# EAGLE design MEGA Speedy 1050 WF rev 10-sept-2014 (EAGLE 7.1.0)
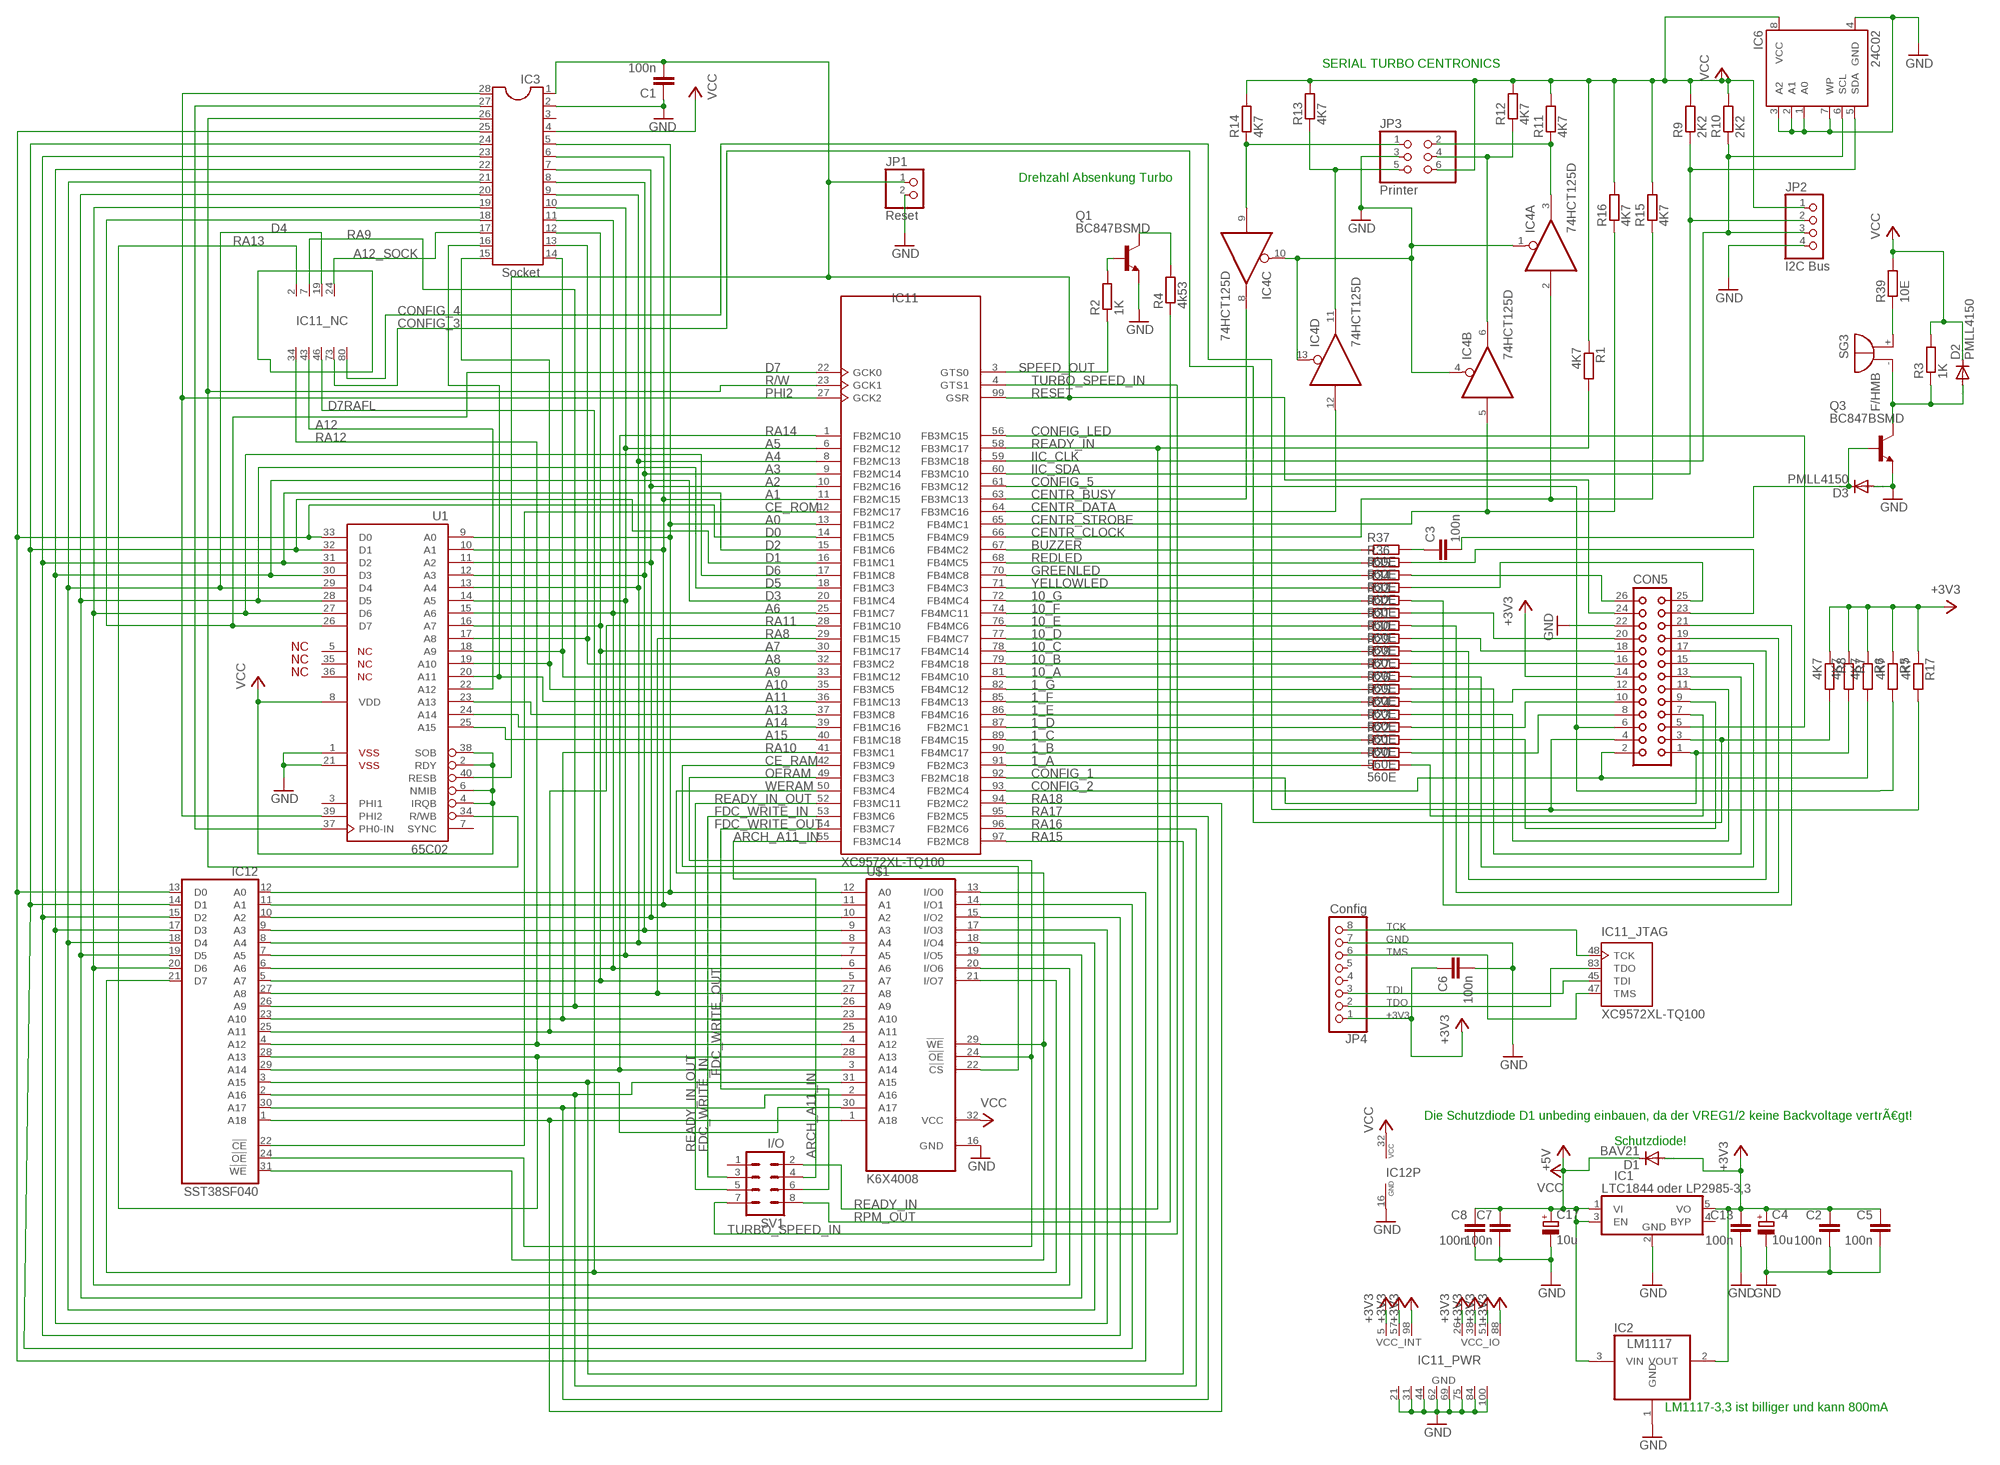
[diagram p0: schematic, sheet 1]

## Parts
C1  100n  C-EUC0805  [C0805]
C2  100n  C-EUC0805  [C0805]
C3  100n  C-EUC0805  [C0805]
C4  10u  CPOL-EUD/7343-31W  [D/7343-31W]
C5  100n  C-EUC0805  [C0805]
C6  100n  C-EUC0805  [C0805]
C7  100n  C-EUC0805  [C0805]
C8  100n  C-EUC0805  [C0805]
C13  100n  C-EUC0805  [C0805]
C17  10u  CPOL-EUD/7343-31W  [D/7343-31W]
CON5  CON26L  [CON26L]
D1  BAV21  PMLL4150  [SOD80C]
D2  PMLL4150  [SOD80C]
D3  PMLL4150  [SOD80C]
IC1  LTC1844 oder LP2985-3,3  LTC1844  [SOT23/5]
IC2  LM1117  REG1117  [SOT223]
IC3  Socket  DIL28  [DIL28-6]
IC4  74HCT125D  [SO14]
IC6  24C02  AT24C  [SOIC8]
IC11  XC9572XL-TQ100  [TQ100]
IC12  SST38SF040  AM29F040J  [PLCC32R]
JP1  Reset  PINHD-1X2  [1X02]
JP2  I2C Bus  PINHD-1X4  [1X04]
JP3  Printer  PINHD-2X3  [2X03]
JP4  Config  PINHD-1X8  [1X08]
Q1  BC847BSMD  [SOT23]
Q3  BC847BSMD  [SOT23]
R1  4K7  R-EU_M0805  [M0805]
R2  1K  R-EU_M0805  [M0805]
R3  1K  R-EU_M0805  [M0805]
R4  4k53  R-EU_M0805  [M0805]
R5  4K7  R-EU_M0805  [M0805]
R6  4K7  R-EU_M0805  [M0805]
R7  4K7  R-EU_M0805  [M0805]
R8  4K7  R-EU_M0805  [M0805]
R9  2K2  R-EU_M0805  [M0805]
R10  2K2  R-EU_M0805  [M0805]
R11  4K7  R-EU_M0805  [M0805]
R12  4K7  R-EU_M0805  [M0805]
R13  4K7  R-EU_M0805  [M0805]
R14  4K7  R-EU_M0805  [M0805]
R15  4K7  R-EU_M0805  [M0805]
R16  4K7  R-EU_M0805  [M0805]
R17  4K7  R-EU_M0805  [M0805]
R20  560E  R-EU_M0805  [M0805]
R21  560E  R-EU_M0805  [M0805]
R22  560E  R-EU_M0805  [M0805]
R23  560E  R-EU_M0805  [M0805]
R24  560E  R-EU_M0805  [M0805]
R25  560E  R-EU_M0805  [M0805]
R26  560E  R-EU_M0805  [M0805]
R27  560E  R-EU_M0805  [M0805]
R28  560E  R-EU_M0805  [M0805]
R29  560E  R-EU_M0805  [M0805]
R30  560E  R-EU_M0805  [M0805]
R31  560E  R-EU_M0805  [M0805]
R32  560E  R-EU_M0805  [M0805]
R33  560E  R-EU_M0805  [M0805]
R34  560E  R-EU_M0805  [M0805]
R35  560E  R-EU_M0805  [M0805]
R36  560E  R-EU_M0805  [M0805]
R37  560E  R-EU_M0805  [M0805]
R39  10E  R-EU_M0805  [M0805]
SG3  F/HMB  [F/HMB]
SV1  I/O  MA04-2  [MA04-2]
U1  65C02  G65SC02P  [DIP-40]
U$1  K6X4008  [SOP32L]

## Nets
1_A: IC11.91(FB2MC3) R20.1
1_B: IC11.90(FB4MC17) R21.1
1_C: IC11.89(FB4MC15) R22.1
1_D: IC11.87(FB2MC1) R23.1
1_E: IC11.86(FB4MC16) R24.1
1_F: IC11.85(FB4MC13) R25.1
1_G: IC11.82(FB4MC12) R26.1
10_A: IC11.81(FB4MC10) R27.1
10_B: IC11.79(FB4MC18) R28.1
10_C: IC11.78(FB4MC14) R29.1
10_D: IC11.77(FB4MC7) R30.1
10_E: IC11.76(FB4MC6) R31.1
10_F: IC11.74(FB4MC11) R32.1
10_G: IC11.72(FB4MC4) R33.1
+3V3: C2.1 C4.+ C5.1 C6.1 C13.1 CON5.14 D1.A IC1.5(VO) IC2.2(VOUT) IC11.5(VCC_INT) IC11.26(VCC_IO) IC11.38(VCC_IO) IC11.51(VCC_IO) IC11.57(VCC_INT) IC11.88(VCC_IO) IC11.98(VCC_INT) JP4.1 R5.1 R6.1 R7.1 R8.1 R17.1
A0: IC3.5 IC11.13(FB1MC2) IC12.12(A0) U1.9(A0) U$1.12(A0)
A1: IC3.6 IC11.11(FB2MC15) IC12.11(A1) U1.10(A1) U$1.11(A1)
A2: IC3.7 IC11.10(FB2MC16) IC12.10(A2) U1.11(A2) U$1.10(A2)
A3: IC3.8 IC11.9(FB2MC14) IC12.9(A3) U1.12(A3) U$1.9(A3)
A4: IC3.9 IC11.8(FB2MC13) IC12.8(A4) U1.13(A4) U$1.8(A4)
A5: IC3.10 IC11.6(FB2MC12) IC12.7(A5) U1.14(A5) U$1.7(A5)
A6: IC3.11 IC11.25(FB1MC7) IC12.6(A6) U1.15(A6) U$1.6(A6)
A7: IC3.12 IC11.30(FB1MC17) IC12.5(A7) U1.16(A7) U$1.5(A7)
A8: IC3.13 IC11.32(FB3MC2) U1.17(A8)
A9: IC3.14 IC11.33(FB1MC12) U1.18(A9)
A10: IC3.15 IC11.35(FB3MC5) U1.19(A10)
A11: IC3.16 IC11.36(FB1MC13) U1.20(A11)
A12: IC11.43(NC) U1.22(A12)
A12_SOCK: IC3.17 IC11.24(NC)
A13: IC11.37(FB3MC8) U1.23(A13)
A14: IC11.39(FB1MC16) U1.24(A14)
A15: IC11.40(FB1MC18) U1.25(A15)
ARCH_A11_IN: IC11.55(FB3MC14) SV1.4
BUZZER: IC11.67(FB4MC2) R37.1
CE_RAM: IC11.42(FB3MC9) U$1.22(!CS)
CE_ROM: IC11.12(FB2MC17) IC12.22(!CE)
CENTR_BUSY: IC4.8(C:O) IC11.63(FB3MC13)
CENTR_CLOCK: IC4.2(A:I) IC11.66(FB4MC9) R15.1
CENTR_DATA: IC4.12(D:I) IC11.64(FB3MC16)
CENTR_STROBE: IC4.5(B:I) IC11.65(FB4MC1) R16.1
CONFIG_1: CON5.1 IC11.92(FB2MC18) R7.2
CONFIG_2: CON5.2 IC11.93(FB2MC4) R6.2
CONFIG_3: CON5.3 IC11.73(NC) R8.2
CONFIG_4: CON5.4 IC11.80(NC) R17.2
CONFIG_5: CON5.6 IC11.61(FB3MC12) R5.2
CONFIG_LED: CON5.5 IC11.56(FB3MC15)
D0: IC3.25 IC11.14(FB1MC5) IC12.13(D0) U1.33(D0) U$1.13(I/O0)
D1: IC3.24 IC11.16(FB1MC1) IC12.14(D1) U1.32(D1) U$1.14(I/O1)
D2: IC3.23 IC11.15(FB1MC6) IC12.15(D2) U1.31(D2) U$1.15(I/O2)
D3: IC3.22 IC11.20(FB1MC4) IC12.17(D3) U1.30(D3) U$1.17(I/O3)
D4: IC3.21 IC11.19(NC) IC12.18(D4) U1.29(D4) U$1.18(I/O4)
D5: IC3.20 IC11.18(FB1MC3) IC12.19(D5) U1.28(D5) U$1.19(I/O5)
D6: IC3.19 IC11.17(FB1MC8) IC12.20(D6) U1.27(D6) U$1.20(I/O6)
D7: IC3.18 IC11.22(GCK0) U1.26(D7)
D7RAFL: IC11.46(NC) IC12.21(D7) U$1.21(I/O7)
FDC_WRITE_IN: IC11.53(FB3MC6) SV1.3
FDC_WRITE_OUT: IC11.54(FB3MC7) SV1.6
GND: C1.1 C2.2 C4.- C5.2 C6.2 C7.2 C8.2 C13.2 C17.- CON5.22 D3.A IC1.2(GND) IC2.1(GND) IC3.2 IC4.1(A:OE) IC4.4(B:OE) IC4.10(C:OE) IC4.13(D:OE) IC6.1(A0) IC6.2(A1) IC6.3(A2) IC6.4(GND) IC6.7(WP) IC11.21(GND) IC11.31(GND) IC11.44(GND) IC11.62(GND) IC11.69(GND) IC11.75(GND) IC11.84(GND) IC11.100(GND) IC12.16(GND) JP1.2 JP2.4 JP3.3 JP4.7 Q1.2(E) Q3.2(E) U1.1(VSS$1) U1.21(VSS$2) U$1.16(GND)
GREENLED: IC11.70(FB4MC8) R35.1
IIC_CLK: IC6.6(SCL) IC11.59(FB3MC18) JP2.3 R10.1
IIC_SDA: IC6.5(SDA) IC11.60(FB3MC10) JP2.2 R9.1
N$2: Q1.1(B) R2.2
N$7: Q1.3(C) R4.2
N$8: R39.1 SG3.+
N$11: D2.A Q3.3(C) R3.1 SG3.-
N$36: IC3.27 U1.37(PH0-IN)
N$41: IC4.6(B:O) JP3.4 R12.1
N$42: IC4.3(A:O) JP3.2 R11.1
N$43: IC4.9(C:I) JP3.1 R14.1
N$44: IC4.11(D:O) JP3.5 R13.1
N$86: C3.1 R37.2
N$96: C3.2 D3.C Q3.1(B)
N$158: CON5.20 R32.2
N$168: CON5.21 R33.2
N$174: CON5.7 R20.2
N$175: CON5.8 R21.2
N$180: CON5.9 R22.2
N$181: CON5.10 R23.2
N$182: CON5.11 R24.2
N$183: CON5.12 R25.2
N$184: CON5.13 R26.2
N$185: CON5.15 R27.2
N$186: CON5.23 R36.2
N$187: CON5.16 R28.2
N$188: CON5.17 R29.2
N$189: CON5.18 R30.2
N$190: CON5.19 R31.2
N$191: CON5.26 R35.2
N$192: CON5.25 R34.2
OERAM: IC11.49(FB3MC3) IC12.24(!OE) U$1.24(!OE)
PHI2: IC3.28 IC11.27(GCK2) U1.39(PHI2)
R/W: IC3.26 IC11.23(GCK1) U1.34(R/WB)
RA8: IC11.29(FB1MC15) IC12.27(A8) U$1.27(A8)
RA9: IC11.7(NC) IC12.26(A9) U$1.26(A9)
RA10: IC11.41(FB3MC1) IC12.23(A10) U$1.23(A10)
RA11: IC11.28(FB1MC10) IC12.25(A11) U$1.25(A11)
RA12: IC11.34(NC) IC12.4(A12) U$1.4(A12)
RA13: IC11.2(NC) IC12.28(A13) U$1.28(A13)
RA14: IC11.1(FB2MC10) IC12.29(A14) U$1.3(A14)
RA15: IC11.97(FB2MC8) IC12.3(A15) U$1.30(A17)
RA16: IC11.96(FB2MC6) IC12.2(A16) U$1.31(A15)
RA17: IC11.95(FB2MC5) IC12.30(A17) U$1.2(A16)
RA18: IC11.94(FB2MC2) IC12.1(A18) U$1.1(A18)
READY_IN: IC11.58(FB3MC17) R1.2 SV1.2
READY_IN_OUT: IC11.52(FB3MC11) SV1.5
REDLED: IC11.68(FB4MC5) R36.1
RESET: C1.2 CON5.24 IC3.1 IC11.99(GSR) JP1.1 U1.40(RESB)
RPM_OUT: R4.1 SV1.8
SPEED_OUT: IC11.3(GTS0) R2.1
TCK: IC11.48(TCK) JP4.8
TDI: IC11.45(TDI) JP4.3
TDO: IC11.83(TDO) JP4.2
TMS: IC11.47(TMS) JP4.6
TURBO_SPEED_IN: IC11.4(GTS1) SV1.7
VCC: C7.1 C8.1 C17.+ D1.C D2.C IC1.1(VI) IC1.3(EN) IC2.3(VIN) IC3.4 IC6.8(VCC) IC12.32(VCC) JP2.1 JP3.6 R1.1 R3.2 R9.2 R10.2 R11.2 R12.2 R13.2 R14.2 R15.2 R16.2 R39.2 U1.2(RDY) U1.4(IRQB) U1.6(NMIB) U1.8(VDD) U1.38(SOB) U$1.32(VCC) ; supply symbol labelled +5V
WERAM: IC11.50(FB3MC4) IC12.31(!WE) U$1.29(!WE)
YELLOWLED: IC11.71(FB4MC3) R34.1
Unconnected: IC1.4(BYP) IC3.3 JP4.4 JP4.5 SV1.1 U1.3(PHI1) U1.5(NC$1) U1.7(SYNC) U1.35(NC$2) U1.36(NC$3)

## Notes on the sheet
- SERIAL TURBO CENTRONICS
- Drehzahl Absenkung Turbo
- Die Schutzdiode D1 unbeding einbauen, da der VREG1/2 keine Backvoltage vertrÃ€gt!
- Schutzdiode!
- LM1117-3,3 ist billiger und kann 800mA

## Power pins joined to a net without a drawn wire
GND: IC4.7(P:GND)
VCC: IC4.14(P:VCC)

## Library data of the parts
C1-C3 C5-C8 C13 = rcl:C-EU: CAPACITOR, European symbol
C4 C17 = rcl:CPOL-EU: POLARIZED CAPACITOR, European symbol
CON5 = con-harting:CON26L: CONNECTOR; OC_FARNELL: unknown; OC_NEWARK: unknown
D1-D3 = diode:PMLL4150: DIODE
IC1 = Sonstiges:LTC1844
IC2 = burr-brown:REG1117: 800mA and 1A Low Dropout (LDO) Positive Regulator 1.8V, 2.5V, 2.85V, 3.3V, 5V, and Adj; MPN: REG1117; OC_FARNELL: 1097566; OC_NEWARK: 14P6981
IC3 = ic-package:DIL28: Dual In Line
IC4 = 74xx-eu:74*125: Quad bus BUFFER, 3-state
IC6 = atmel:AT24C*: 2-wire serial EEPROM
IC11 = XC9500XLneu_wf:XC9572XL-TQ100
IC12 = am29-memory:AM29F040J: 4-Megabit FLASH MEMORY (512 K x 8 bit) 5 V-only
JP1 = pinhead:PINHD-1X2: PIN HEADER
JP2 = pinhead:PINHD-1X4: PIN HEADER
JP3 = pinhead:PINHD-2X3: PIN HEADER
JP4 = pinhead:PINHD-1X8: PIN HEADER
Q1 Q3 = transistor-npn:BC847*: NPN Transistor
R1-R17 R20-R37 R39 = rcl:R-EU_: RESISTOR, European symbol
SG3 = buzzer:F/HMB: BUZZER; OC_FARNELL: unknown; OC_NEWARK: unknown
SV1 = con-lstb:MA04-2: PIN HEADER; OC_FARNELL: unknown; OC_NEWARK: unknown
U1 = 65xxx:G65SC02P: California Micro Devices Version
U$1 = memory:K6X4008

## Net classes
2 3.3: width 0.508 mm, clearance 0.254 mm

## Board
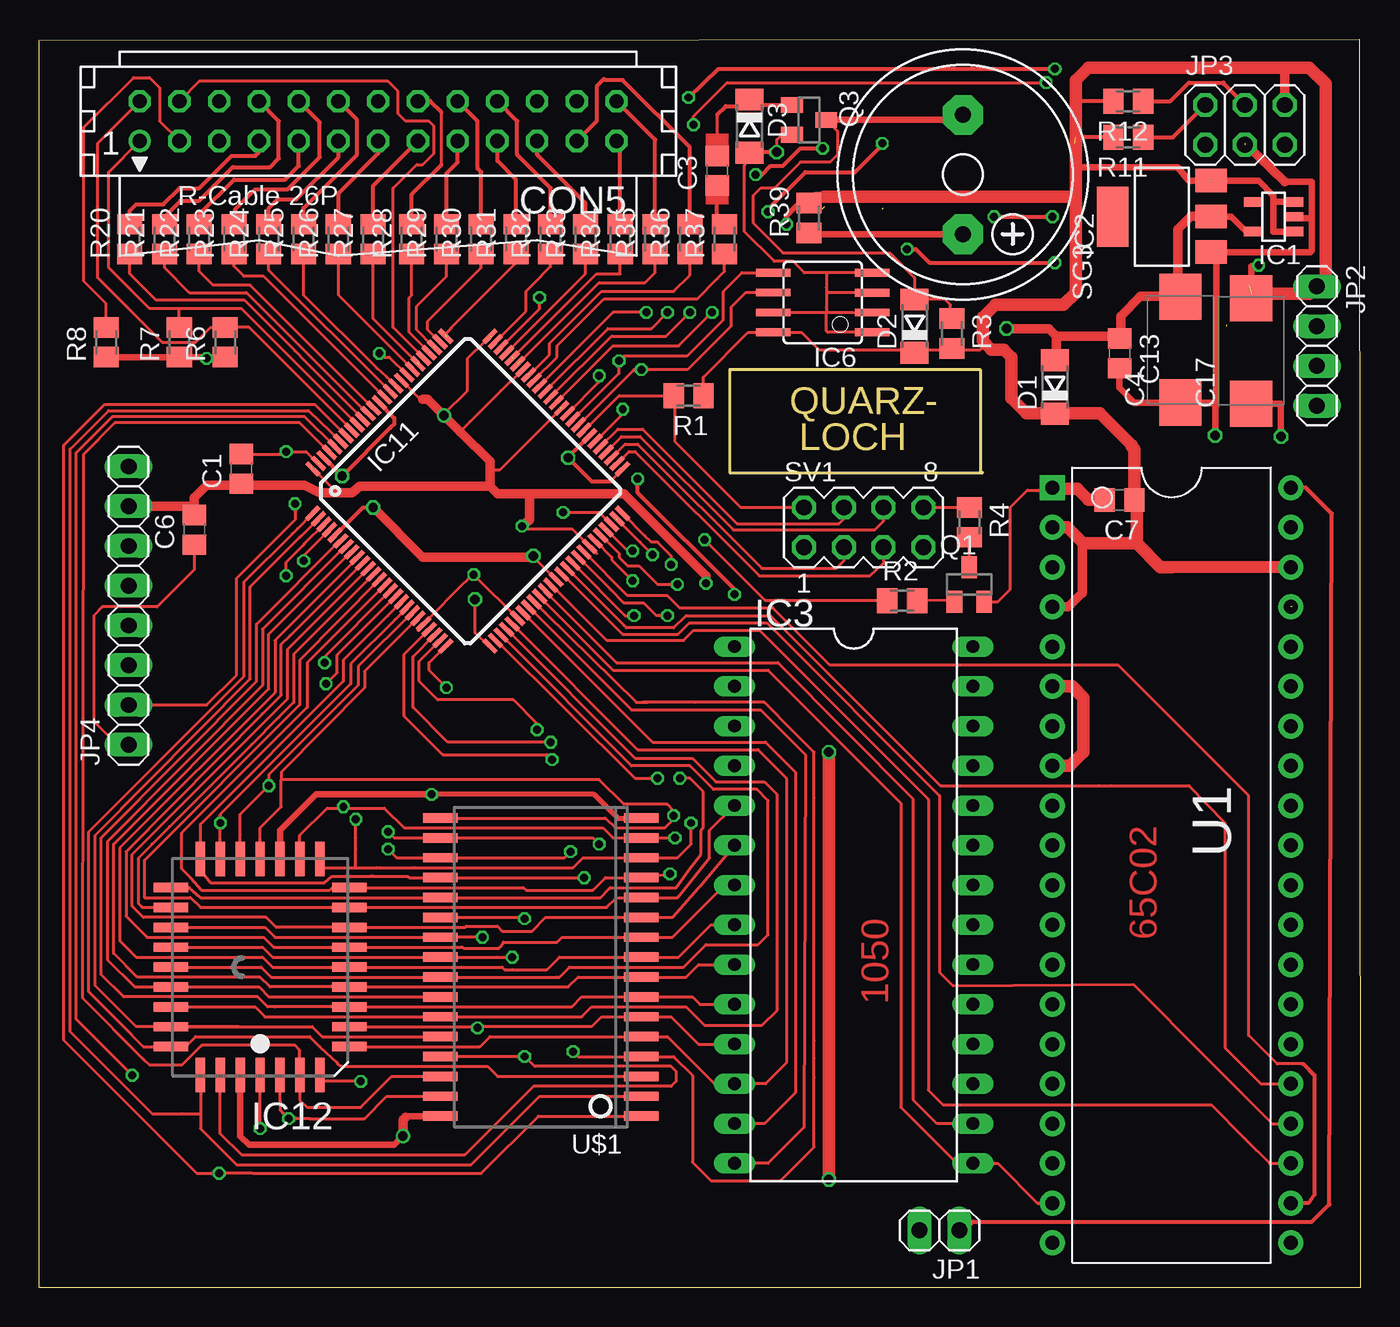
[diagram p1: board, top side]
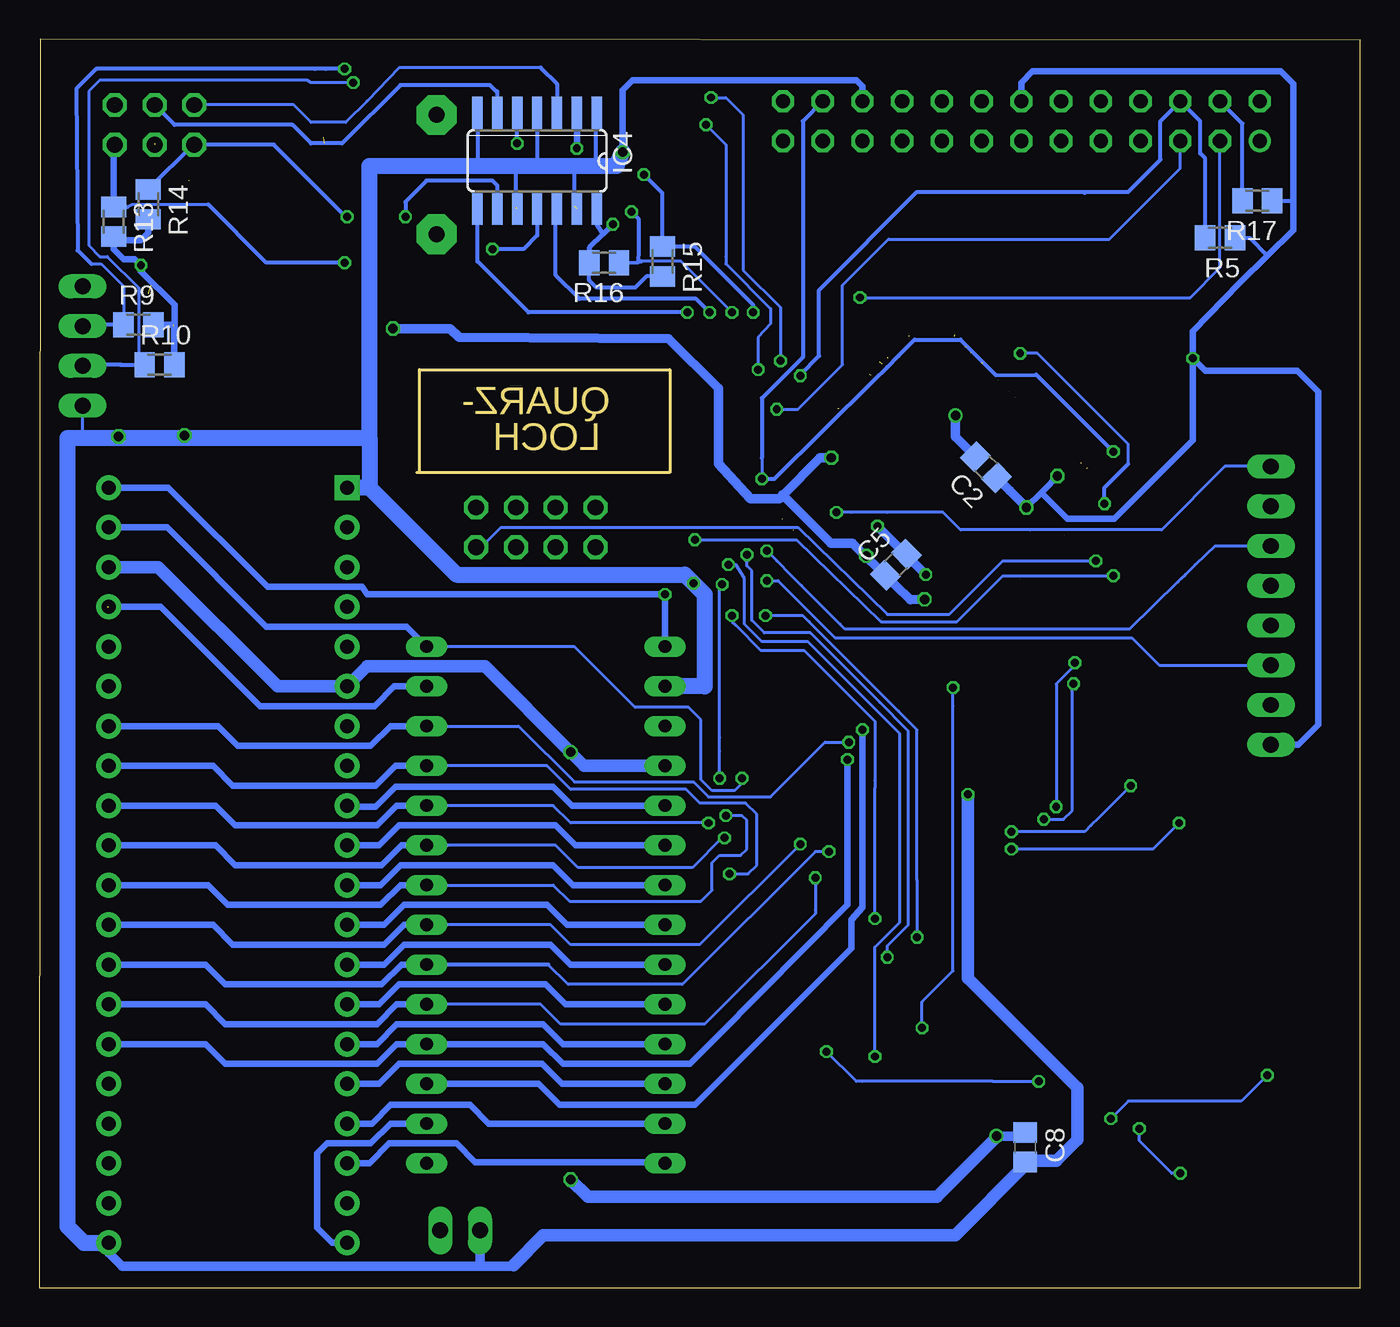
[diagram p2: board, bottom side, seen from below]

Size 84.46 x 79.77 mm. Coordinates in mm from the lower left corner, seen from the top.
Outline: 0,0 0,79.69 84.38,79.77 84.46,0 0,0
Copper layers (1*16): Top 0.035mm / dielectric 1.5mm / Bottom 0.035mm
Design rules "ITEADstudio_DRC": minimum track width 6mil, minimum drill 12mil, track to track 6mil, track to pad 6mil, pad to pad 6mil, via to via 6mil, smd to smd 0mil, copper to edge 10mil, drill to drill 10mil, minimum pad ring 10mil, minimum via ring 6mil, stop-mask expansion 2mil, vias tented up to drill 100mil, thermal gap 10mil
Milling: 4 lines

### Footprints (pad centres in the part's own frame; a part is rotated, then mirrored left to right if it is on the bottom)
C0805 = smd 1.3 x 1.5: 1 -0.95,0; 2 0.95,0
D/7343-31W = smd 2.95 x 2.7: + 3.375,0; - -3.375,0
CON26L = drill 0.914: 1 15.24,1.27 | drill 0.914 octagon: 2 15.24,-1.27; 3 12.7,1.27; 4 12.7,-1.27; 5 10.16,1.27; 6 10.16,-1.27; 7 7.62,1.27; 8 7.62,-1.27; 9 5.08,1.27; 10 5.08,-1.27; 11 2.54,1.27; 12 2.54,-1.27; 13 0,1.27; 14 0,-1.27; 15 -2.54,1.27; 16 -2.54,-1.27; 17 -5.08,1.27; 18 -5.08,-1.27; 19 -7.62,1.27; 20 -7.62,-1.27; 21 -10.16,1.27; 22 -10.16,-1.27; 23 -12.7,1.27; 24 -12.7,-1.27; 25 -15.24,1.27; 26 -15.24,-1.27
SOD80C = smd 1.4 x 1.8: A 1.7,0; C -1.7,0
SOT23/5 = smd 0.6 x 1.2: 1 -0.95,-1.306; 2 0,-1.306; 3 0.95,-1.306; 4 0.95,1.306; 5 -0.95,1.306
SOT223 = smd 1.499 x 2.007: 1 -2.261,-3.15; 2 0.025,-3.15; 3 2.311,-3.15 | smd 3.81 x 2.007: 4 0,3.15
DIL28-6 = drill 0.813 long: 1 -16.51,-7.62; 2 -13.97,-7.62; 3 -11.43,-7.62; 4 -8.89,-7.62; 5 -6.35,-7.62; 6 -3.81,-7.62; 7 -1.27,-7.62; 8 1.27,-7.62; 9 3.81,-7.62; 10 6.35,-7.62; 11 8.89,-7.62; 12 11.43,-7.62; 13 13.97,-7.62; 14 16.51,-7.62; 15 16.51,7.62; 16 13.97,7.62; 17 11.43,7.62; 18 8.89,7.62; 19 6.35,7.62; 20 3.81,7.62; 21 1.27,7.62; 22 -1.27,7.62; 23 -3.81,7.62; 24 -6.35,7.62; 25 -8.89,7.62; 26 -11.43,7.62; 27 -13.97,7.62; 28 -16.51,7.62
SO14 = smd 0.66 x 2.032: 1 -3.81,-3.073; 2 -2.54,-3.073; 3 -1.27,-3.073; 4 0,-3.073; 5 1.27,-3.073; 6 2.54,-3.073; 7 3.81,-3.073; 8 3.81,3.073; 9 2.54,3.073; 10 1.27,3.073; 11 0,3.073; 12 -1.27,3.073; 13 -2.54,3.073; 14 -3.81,3.073
SOIC8 = smd 0.5 x 2.2: 1 -1.905,-3.154; 2 -0.645,-3.154; 3 0.625,-3.154; 4 1.895,-3.154; 5 1.905,3.154; 6 0.635,3.154; 7 -0.635,3.154; 8 -1.905,3.154
TQ100 = smd 1.118 x 0.305: 1 -8,6; 2 -8,5.5; 3 -8,5; 4 -8,4.5; 5 -8,4; 6 -8,3.5; 7 -8,3; 8 -8,2.5; 9 -8,2; 10 -8,1.5; 11 -8,1; 12 -8,0.5; 13 -8,0; 14 -8,-0.5; 15 -8,-1; 16 -8,-1.5; 17 -8,-2; 18 -8,-2.5; 19 -8,-3; 20 -8,-3.5; 21 -8,-4; 22 -8,-4.5; 23 -8,-5; 24 -8,-5.5; 25 -8,-6; 51 8,-6; 52 8,-5.5; 53 8,-5; 54 8,-4.5; 55 8,-4; 56 8,-3.5; 57 8,-3; 58 8,-2.5; 59 8,-2; 60 8,-1.5; 61 8,-1; 62 8,-0.5; 63 8,0; 64 8,0.5; 65 8,1; 66 8,1.5; 67 8,2; 68 8,2.5; 69 8,3; 70 8,3.5; 71 8,4; 72 8,4.5; 73 8,5; 74 8,5.5; 75 8,6 | smd 0.305 x 1.118: 26 -6,-8; 27 -5.5,-8; 28 -5,-8; 29 -4.5,-8; 30 -4,-8; 31 -3.5,-8; 32 -3,-8; 33 -2.5,-8; 34 -2,-8; 35 -1.5,-8; 36 -1,-8; 37 -0.5,-8; 38 0,-8; 39 0.5,-8; 40 1,-8; 41 1.5,-8; 42 2,-8; 43 2.5,-8; 44 3,-8; 45 3.5,-8; 46 4,-8; 47 4.5,-8; 48 5,-8; 49 5.5,-8; 50 6,-8; 76 6,8; 77 5.5,8; 78 5,8; 79 4.5,8; 80 4,8; 81 3.5,8; 82 3,8; 83 2.5,8; 84 2,8; 85 1.5,8; 86 1,8; 87 0.5,8; 88 0,8; 89 -0.5,8; 90 -1,8; 91 -1.5,8; 92 -2,8; 93 -2.5,8; 94 -3,8; 95 -3.5,8; 96 -4,8; 97 -4.5,8; 98 -5,8; 99 -5.5,8; 100 -6,8
PLCC32R = smd 0.6 x 2.2: 1 0,6.9; 2 -1.27,6.9; 3 -2.54,6.9; 4 -3.81,6.9; 14 -3.81,-6.9; 15 -2.54,-6.9; 16 -1.27,-6.9; 17 0,-6.9; 18 1.27,-6.9; 19 2.54,-6.9; 20 3.81,-6.9; 30 3.81,6.9; 31 2.54,6.9; 32 1.27,6.9 | smd 2.2 x 0.6: 5 -5.7,5.08; 6 -5.7,3.81; 7 -5.7,2.54; 8 -5.7,1.27; 9 -5.7,0; 10 -5.7,-1.27; 11 -5.7,-2.54; 12 -5.7,-3.81; 13 -5.7,-5.08; 21 5.7,-5.08; 22 5.7,-3.81; 23 5.7,-2.54; 24 5.7,-1.27; 25 5.7,0; 26 5.7,1.27; 27 5.7,2.54; 28 5.7,3.81; 29 5.7,5.08
1X02 = drill 1.016 long: 1 -1.27,0; 2 1.27,0
1X04 = drill 1.016 long: 1 -3.81,0; 2 -1.27,0; 3 1.27,0; 4 3.81,0
2X03 = drill 1.016 octagon: 1 -2.54,-1.27; 2 -2.54,1.27; 3 0,-1.27; 4 0,1.27; 5 2.54,-1.27; 6 2.54,1.27
1X08 = drill 1.016 long: 1 -8.89,0; 2 -6.35,0; 3 -3.81,0; 4 -1.27,0; 5 1.27,0; 6 3.81,0; 7 6.35,0; 8 8.89,0
SOT23 = smd 1 x 1.4: 1 -0.95,-1.1; 2 0.95,-1.1; 3 0,1.1
M0805 = smd 1.3 x 1.6: 1 -0.95,0; 2 0.95,0
F/HMB = drill 1.016 pad 2.54 octagon: + 3.81,0; - -3.81,0
MA04-2 = drill 1.016 octagon: 1 -3.81,-1.27; 2 -3.81,1.27; 3 -1.27,-1.27; 4 -1.27,1.27; 5 1.27,-1.27; 6 1.27,1.27; 7 3.81,-1.27; 8 3.81,1.27
DIP-40 = drill 0.889 pad 1.6 square: 1 -22.86,-7.62 | drill 0.889 pad 1.6: 2 -20.32,-7.62; 3 -17.78,-7.62; 4 -15.24,-7.62; 5 -12.7,-7.62; 6 -10.16,-7.62; 7 -7.62,-7.62; 8 -5.08,-7.62; 9 -2.54,-7.62; 10 0,-7.62; 11 2.54,-7.62; 12 5.08,-7.62; 13 7.62,-7.62; 14 10.16,-7.62; 15 12.7,-7.62; 16 15.24,-7.62; 17 17.78,-7.62; 18 20.32,-7.62; 19 22.86,-7.62; 20 25.4,-7.62; 21 25.4,7.62; 22 22.86,7.62; 23 20.32,7.62; 24 17.78,7.62; 25 15.24,7.62; 26 12.7,7.62; 27 10.16,7.62; 28 7.62,7.62; 29 5.08,7.62; 30 2.54,7.62; 31 0,7.62; 32 -2.54,7.62; 33 -5.08,7.62; 34 -7.62,7.62; 35 -10.16,7.62; 36 -12.7,7.62; 37 -15.24,7.62; 38 -17.78,7.62; 39 -20.32,7.62; 40 -22.86,7.62
SOP32L = smd 0.6 x 2.2: 1 -9.525,-6.416; 2 -8.255,-6.416; 3 -6.985,-6.416; 4 -5.715,-6.416; 5 -4.445,-6.416; 6 -3.175,-6.416; 7 -1.905,-6.416; 8 -0.635,-6.416; 9 0.635,-6.416; 10 1.905,-6.416; 11 3.175,-6.416; 12 4.445,-6.416; 13 5.715,-6.416; 14 6.985,-6.416; 15 8.255,-6.416; 16 9.525,-6.416; 17 9.525,6.416; 18 8.255,6.416; 19 6.985,6.416; 20 5.715,6.416; 21 4.445,6.416; 22 3.175,6.416; 23 1.905,6.416; 24 0.635,6.416; 25 -0.635,6.416; 26 -1.905,6.416; 27 -3.175,6.416; 28 -4.445,6.416; 29 -5.715,6.416; 30 -6.985,6.416; 31 -8.255,6.416; 32 -9.525,6.416

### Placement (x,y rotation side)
C1  12.94,52.31 90 top
C2  23.93,52.41 135 bottom
C3  43.34,71.36 90 top
C4  72.95,59.93 90 top
C5  29.69,46.2 45 bottom
C6  9.92,48.42 90 top
C7  69.06,50.32 180 top
C8  21.43,8.97 270 bottom
C13  69.06,59.69 270 top
C17  77.47,59.85 90 top
CON5  21.67,74.53 180 top
D1  64.93,57.55 90 top
D2  55.96,61.44 90 top
D3  45.4,74.22 270 top
IC1  78.9,68.42 90 top
IC2  71.76,68.42 90 top
IC3  52.07,24.45 270 top
IC4  52.63,71.99 180 bottom
IC6  50.09,62.94 90 top
IC11  27.4,50.89 45 top
IC12  14.13,20.48 180 top
JP1  57.55,3.65 180 top
JP2  81.68,60.17 270 top
JP3  77.07,74.3 0 top
JP4  5.72,43.58 90 top
Q1  59.45,44.93 0 top
Q3  49.21,74.61 270 top
R1  41.51,56.99 180 top
R2  55.17,43.89 0 top
R3  58.34,60.96 270 top
R4  59.45,48.9 270 top
R5  8.97,67.07 180 bottom
R6  11.91,60.4 90 top
R7  8.97,60.4 90 top
R8  4.29,60.4 90 top
R9  78.1,61.52 0 bottom
R10  76.76,58.98 0 bottom
R11  69.61,73.5 180 top
R12  69.61,75.8 180 top
R13  79.69,68.1 270 bottom
R14  77.47,69.22 270 bottom
R15  44.61,65.56 270 bottom
R16  48.34,65.48 180 bottom
R17  6.59,69.45 180 bottom
R20  5.79,66.99 90 top
R21  8.02,66.99 90 top
R22  10.24,66.99 90 top
R23  12.46,66.99 90 top
R24  14.68,66.99 90 top
R25  16.91,66.99 90 top
R26  19.13,66.99 90 top
R27  21.35,66.99 90 top
R28  23.81,66.99 90 top
R29  26.04,66.99 90 top
R30  28.26,66.99 90 top
R31  30.48,66.99 90 top
R32  32.7,66.99 90 top
R33  34.93,66.99 90 top
R34  37.15,66.99 90 top
R35  39.37,66.99 90 top
R36  41.59,66.99 90 top
R37  43.82,66.99 90 top
R39  49.21,68.34 90 top
SG3  59.05,71.12 270 top
SV1  52.71,48.58 0 top
U1  72.39,28.26 270 top
U$1  32.07,20.48 90 top

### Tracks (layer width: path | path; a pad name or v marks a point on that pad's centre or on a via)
1_A
  Top 0.203: IC11.91 20.68,55.52 16.99,59.21 16.35,59.85 13.1,63.1 7.46,63.1 5.79,64.77 | 5.79,64.77 | 6.03,66.36 R20.1 5.79,64.77
1_B
  Top 0.203: IC11.90 20.99,55.84 13.26,63.58 9.6,63.58 8.02,65.17 R21.1
1_C
  Top 0.203: IC11.89 21.35,56.2 13.49,64.06 11.11,64.06 10.24,64.93 R22.1
1_D  (1 unrouted)
  Top 0.203: 22.09,56.88 14.37,64.61 13.1,64.61 12.46,65.25 R23.1
1_E  (1 unrouted)
  Top 0.203: 22.44,57.26 14.68,65.01 R24.1
1_F
  Top 0.203: IC11.85 22.24,58.17 21.91,58.48 21.59,58.74 16.91,63.42 R25.1
1_G
  Top 0.203: IC11.82 23.86,58.69 19.13,63.42 R26.1 19.37,66.36
10_A  (1 unrouted)
  Top 0.203: 24.16,59.1 21.35,61.91 R27.1
10_B  (1 unrouted)
  Top 0.203: 24.92,59.77 23.65,61.04 23.65,63.26 23.81,63.42 R28.1
10_C  (1 unrouted)
  Top 0.203: 25.2,60.13 24.13,61.2 24.13,62.71 26.04,64.61 R29.1
10_D
  Top 0.203: IC11.77 25.6,60.44 24.84,61.2 24.84,61.75 27.54,64.45 28.26,65.17 R30.1
10_E  (1 unrouted)
  Top 0.203: 25.96,60.87 26.35,61.36 28.18,63.18 30.48,65.48 R31.1
10_F
  Top 0.203: R32.1 32.39,66.04 32.7,65.72 32.7,65.25 31.59,64.14 31.12,63.66 31.12,62.39 IC11.74
10_G
  Top 0.203: IC11.72 29.89,59.73 34.93,64.77 34.93,65.72 34.61,66.04 R33.1
+3V3  (via drill 0.51, 0.6)  (1 unrouted)
  Top 0.203: 36.51,51.51 37.3,52.3 | 28.78,40.99 27.86,41.83 v27.86,43.97 | IC11.38 33.06,45.29 32.98,45.29 31.59,46.67 v31.59,46.75 | C6.1 9.92,45.88 7.54,43.5 4.05,43.5 3.49,42.94 3.49,36.2 5,34.69 JP4.1
  Top 0.254: IC11.98 v19.37,51.85 22.44,54.93 22.7,55.17 22.7,55.56 21.74,56.52 IC11.88 | IC11.57 34.09,53.34 v33.81,53.02 35.32,51.51 36.51,51.51 | 37.3,52.3 IC11.51 | IC11.26 28.78,40.99 | 18.93,48.06 20.72,49.85 v21.35,49.85
  Top 0.406: IC1.5 77.15,67.47 76.2,68.42 74.93,68.42 IC2.2 | IC2.2 74.85,68.5 | IC2.2 | v10.72,59.37 v10.72,59.38 11.83,59.38 R6.1 | R6.1 | R6.1 R7.1 R8.1
  Top 0.61: 72.91,63.34 72.79,63.46 72.79,67.63 73.61,68.45 IC2.2 | 65.01,60.8 64.53,61.28 v61.83,61.28 | 31.59,46.67 24.53,46.67 v21.35,49.85 | 65.01,60.8 65.01,59.33 D1.A | 65.01,60.8 68.63,60.8 C13.1 69.14,61.17 69.14,62.07 70.41,63.34 72.91,63.34 | 72.91,63.34 C4.+
  Bottom 0.203: 10.72,61.12 10.72,61.04 v10.72,59.37 | 10.71,58.58 10.72,58.58 | C5.1 30.36,45.45 28.77,43.93
  Bottom 0.254: 19.21,51.99 v19.37,51.85 | 31.71,46.79 v31.59,46.75 | R17.1 4.29,69.45 | R5.1 7.07,67.07 5.94,65.94
  Bottom 0.406: v21.35,49.85 20.4,50.8 | 20.4,50.8 19.21,51.99 | 20.4,50.8 18.73,49.13 15.72,49.13 10.72,54.13 10.72,58.58 10.72,61.04 | CON5.14 21.67,76.99 20.96,77.71 11.67,77.71 5.08,77.71 4.29,76.91 4.29,69.45 4.29,67.55 5.94,65.94 7.7,64.21 10.72,61.12 | JP4.1 3.97,34.69 2.7,35.96 2.7,57.23 4.05,58.58 9.92,58.58 v10.72,59.37
  Bottom 0.61: C2.1 22.41,50.9 v21.35,49.85 | 36.93,50.65 37.15,50.4 38.97,50.4 41.04,52.63 41.04,57.47 44.21,60.64 57.63,60.72 58.18,61.28 v61.83,61.28 | 36.93,50.65 36.91,50.64 34.53,53.02 v33.81,53.02 | v27.86,43.97 28.77,43.93 31.71,46.79 32.46,47.55 33.83,47.55 36.93,50.65
A0  (1 unrouted)
  Top 0.203: IC3.5 42.86,29.21 42.86,27.46 40.8,24.92 U$1.12 36.91,24.92 36.27,24.29 32.54,24.29 32.23,24.29 IC12.12 10.32,24.29 9.68,24.92 6.75,24.92 6.75,27.3 16.67,37.23 16.67,40.08 IC11.13
  Bottom 0.254: 64.69,30.72 U1.9
  Bottom 0.406: IC3.5 50.4,30.8 51.59,31.99 61.67,31.99 62.94,30.72 64.69,30.72
A1
  Top 0.203: IC3.6 42.23,25.64 42.15,25.56 40.48,23.65 U$1.11 32.39,23.65 31.51,22.78 29.61,22.78 29.29,23.1 27.31,23.1 27.23,23.02 IC12.11 15.32,23.02 15.16,23.02 14.53,23.65 6.67,23.65 5.95,24.37 5.95,27.7 15.88,37.62 15.88,40.78 IC11.11
  Bottom 0.406: U1.10 62.71,28.26 61.44,29.53 51.44,29.53 50.17,28.26 45.64,28.26 44.85,28.26 IC3.6
A2
  Top 0.203: IC3.7 44.29,25.72 43.82,25.72 40.48,22.38 U$1.10 33.42,22.38 33.1,22.07 29.69,22.07 29.45,21.75 | 29.45,21.75 29.37,21.67 27.15,21.67 27.07,21.75 26.99,21.75 IC12.10 15,21.75 14.37,22.38 6.91,22.38 6.11,23.18 5.56,23.73 5.56,27.86 14.29,36.67 15.48,37.86 15.48,41.12 16.03,41.65 IC11.10 | 29.45,21.75
  Bottom 0.406: U1.11 62.63,25.72 61.36,26.99 51.59,26.99 50.32,25.72 IC3.7
A3
  Top 0.203: IC3.8 44.61,23.18 42.94,23.18 40.88,21.11 U$1.9 33.26,21.11 32.46,20.32 30.24,20.32 29.77,20.32 29.61,20.48 26.99,20.48 IC12.9 14.92,20.48 14.29,21.11 6.19,21.11 5.16,22.15 5.16,28.1 15.08,38.02 15.08,41.35 20.33,46.6 IC11.9
  Bottom 0.406: U1.12 62.39,23.18 61.12,24.45 51.99,24.45 50.72,23.18 45.72,23.18 45.01,23.18 IC3.8
A4
  Top 0.203: IC3.9 44.13,20.64 43.34,20.64 42.15,20.64 41.35,19.84 U$1.8 34.45,19.84 33.81,19.21 IC12.8 14.76,19.21 14.13,19.84 6.27,19.84 4.76,21.35 4.76,28.34 14.68,38.26 14.68,41.75 19.94,47 IC11.8
  Bottom 0.406: U1.13 62.39,20.64 61.12,21.91 51.75,21.91 50.48,20.64 IC3.9
A5
  Top 0.203: IC3.10 42.23,18.1 41.75,18.57 U$1.7 34.69,18.57 34.05,17.94 IC12.7 15.08,17.94 14.61,17.94 13.97,18.57 5.4,18.57 3.97,20 3.97,28.73 13.89,38.73 13.89,42.39 19.22,47.71 IC11.6
  Bottom 0.406: U1.14 62.71,18.1 61.44,19.37 52.07,19.37 50.8,18.1 IC3.10 44.29,18.1
A6  (via drill 0.51)
  Top 0.203: IC3.11 44.29,15.56 42.15,15.56 40.4,17.3 U$1.6 35.96,17.3 35.32,16.67 28.1,16.67 v28.02,16.59 27.94,16.67 IC12.6 | IC11.25 25.91,40.91 24.92,39.93 | v26.04,38.34 24.92,39.45 24.92,39.93 | 24.92,39.93
  Bottom 0.203: v28.02,16.59 28.02,18.26 26.04,20.24 26.04,37.15 v26.04,38.34
  Bottom 0.406: U1.15 62.87,15.56 61.6,16.83 52.23,16.83 50.96,15.56 IC3.11
A7
  Top 0.203: IC12.5 28.18,15.4 28.81,16.03 U$1.5 | U$1.5 | U$1.5 40.16,16.03 43.18,13.02 IC3.12 46.43,13.02 47.78,14.37 47.78,32.54 45.96,34.37 38.26,34.37 IC11.30
  Bottom 0.406: U1.16 62.71,13.02 61.44,14.29 52.31,14.29 51.04,13.02 44.61,13.02 45.09,13.02 IC3.12
A8
  Top 0.203: IC11.32 39.21,34.85 46.43,34.85 48.34,32.94 48.34,12.46 46.36,10.48 IC3.13
  Bottom 0.406: U1.17 63.18,10.48 61.99,11.67 56.91,11.67 55.72,10.48 IC3.13
A9
  Top 0.203: IC3.14 46.59,7.94 48.9,10.24 48.97,34.05 46.12,36.91 37.86,36.91 31.3,43.47 IC11.33
  Bottom 0.203: 44.53,8.02 IC3.14
  Bottom 0.406: U1.18 63.34,7.94 62.07,9.21 57.79,9.21 56.59,8.02 44.53,8.02
A10
  Top 0.203: IC11.35 31.99,44.13 36.67,39.45 46.59,39.45 55.09,30.96 55.09,11.51 58.66,7.94 IC3.15 61.28,7.94 63.82,5.4 U1.19
A11
  Top 0.203: IC3.16 57.39,10.48 55.88,11.99 55.88,31.19 47.23,39.93 36.91,39.93 32.39,44.45 32.39,44.53 IC11.36
  Bottom 0.254: 64.69,2.86 U1.20
  Bottom 0.406: IC3.16 61.99,10.48 63.26,9.21 66.04,9.21 66.68,8.57 66.68,3.81 65.72,2.86 U1.20
A12
  Top 0.203: 80.8,14.29 79.14,14.29 77.31,16.11 77.31,31.43 68.98,39.77 50.56,39.77 46.91,43.42 40.96,43.42 40.16,44.21 37.61,44.21 IC11.43
  Top 0.254: 80.8,14.29 81.52,13.57 81.52,5.95 81.12,5.4 U1.22
A12_SOCK  (via drill 0.51)
  Top 0.203: v31.83,35.64 31.83,36.04 30.32,37.54 25.48,37.54 24.29,38.73 24.29,40.01 IC11.24
  Bottom 0.406: IC3.17 52.55,13.02 51.2,11.67 42.55,11.67 32.54,21.67 32.54,23.5 31.83,24.29 v31.83,35.64
A13
  Top 0.203: IC11.37 32.75,44.88 36.27,41.35 41.2,41.35 41.83,41.99 46.04,41.99 56.83,31.19 56.83,12.62 57.79,11.67 74.93,11.67 77.07,9.53 78.66,7.94 U1.23
A14
  Top 0.203: U1.24 78.82,10.48 74.69,14.61 69.93,19.37 58.42,19.29 57.55,20.16 57.55,31.43 46.51,42.47 41.56,42.47 40.85,41.75 37.31,41.75 33.47,45.59 IC11.39
A15
  Top 0.203: U1.25 78.11,13.02 75.8,15.32 75.8,29.69 73.5,32.07 68.5,32.07 67.71,32.07 57.63,32.07 46.75,42.94 41.35,42.94 40.56,42.15 37.54,42.15 37.39,42.31 | IC11.40 37.39,42.31 | 37.39,42.31
ARCH_A11_IN
  Top 0.203: IC11.55 35.88,53.74 36.99,54.85 38.58,54.85 44.61,48.82 51.12,48.82 51.44,49.13 SV1.4
BUZZER
  Top 0.203: IC11.67 31.64,57.99 33.1,59.45 33.1,60.17 36.12,63.18 42.07,63.18 43.34,64.45 43.82,64.93 R37.1
CE_RAM  (via drill 0.51)
  Top 0.203: IC11.42 34.45,46.67 | IC11.42 | v31.04,23.57 30.96,23.65 30.64,23.65 U$1.22 | v40.16,42.94 39.45,42.94 38.66,43.74 37.39,43.74 36.51,44.61 IC11.42
  Bottom 0.203: v31.04,23.57 31.04,23.65 31.04,23.89 31.04,31.91 31.04,32.38 31.04,36.2 35.56,40.72 38.34,40.72 39.93,42.31 40.16,42.55 v40.16,42.94
CE_ROM
  Top 0.203: IC12.22 6.59,24.29 6.35,24.53 6.35,27.46 7.22,28.34 8.33,29.45 11.35,32.46 13.57,34.69 15.32,36.43 16.27,37.39 16.27,39.05 16.28,40.48 IC11.12
CENTR_BUSY  (via drill 0.51)
  Top 0.203: IC11.63 | IC11.63 36.67,60.17 40.88,60.17 v43.02,62.31
  Bottom 0.254: v43.02,62.31 53.18,62.31 56.44,65.56 IC4.8
CENTR_CLOCK  (via drill 0.51)
  Top 0.203: v38.81,62.31 36.69,62.31 IC11.66
  Top 0.254: v45.8,71.12 46.2,71.12 46.75,71.68 47.55,71.68 48.66,72.79 v50.09,72.79
  Bottom 0.254: v45.8,71.12 44.61,69.93 R15.1 44.37,66.52 42.55,66.52 38.81,62.79 v38.81,62.31
  Bottom 0.406: v50.09,72.79 IC4.2
CENTR_DATA  (via drill 0.51)
  Top 0.203: IC11.64 32.7,56.91 36.59,60.8 40.08,60.8 v41.59,62.31
  Bottom 0.254: v41.59,62.31 42.47,63.18 49.93,63.18 51.44,64.69 51.44,68.84 IC4.12
CENTR_STROBE  (via drill 0.51)
  Top 0.203: IC11.65 32.35,57.27 36.35,61.28 39.13,61.28 v40.16,62.31
  Top 0.254: v46.59,68.74 46.59,68.9 48.97,71.28 52.15,71.28 53.9,73.03 v53.9,73.1
  Bottom 0.203: 45.96,65.56 43.42,65.56 v40.16,62.31
  Bottom 0.254: 45.96,65.56 46.16,65.52 | 46.16,65.52 46.12,66.28 46.12,68.26 v46.59,68.74 | v53.9,73.1 IC4.5 | R16.1 46.16,65.52
CONFIG_1
  Top 0.203: IC11.92 20.33,55.16 12.94,62.55 8.97,62.55 | CON5.1 4.45,71.28 4.45,65.17 7.06,62.55 8.97,62.55 | R7.2 8.97,62.55 | 8.97,62.55
CONFIG_2
  Top 0.203: IC11.93 19.97,54.8 13.41,61.36 R6.2 10.95,61.36 10,60.4 7.86,60.4 3.73,64.53 3.73,73.1 CON5.2
CONFIG_3  (via drill 0.51)
  Top 0.203: IC11.73 31.99,62.55 v31.99,63.26 | R8.2 4.29,62.87 2.86,64.29 2.86,74.14 6.03,77.31 7.06,77.31 7.7,76.68 7.7,74.53 CON5.3
  Bottom 0.203: v31.99,63.26 10.87,63.26 8.97,65.17 CON5.3
CONFIG_4
  Top 0.203: IC11.80 24.57,59.41 22.62,61.36 22.62,70.25 24.13,71.75 24.53,71.75 25.24,72.47 25.24,74.22 24.92,74.53 23.42,74.53 22.94,75.01 22.94,76.44 22.3,77.07 10.24,77.07 CON5.4
  Bottom 0.254: R17.2 7.54,74.37 CON5.4
CONFIG_5  (via drill 0.51)
  Top 0.203: IC11.61 35.8,57.86 v35.8,58.26
  Bottom 0.203: v35.8,58.26 35.8,58.34 | 14.92,70.01 14.84,70.01
  Bottom 0.254: 35.8,58.34 34.61,59.53 34.61,63.74 28.34,70.01 17.7,70.01 | 17.7,70.01 14.92,70.01 | 14.84,70.01 12.78,72.07 12.78,74.53 CON5.6 10.24,74.53 10.24,72.47 9.92,72.15 R5.2 | 17.62,69.93 17.7,70.01
CONFIG_LED  (via drill 0.51)
  Top 0.203: IC11.56 35.58,54.08 37.31,55.8 v37.31,56.12
  Bottom 0.203: v37.31,56.12 35.96,56.12 33.1,58.98 33.1,64.06 30.16,66.99 16.03,66.99 11.51,71.52 CON5.5
D0  (via drill 0.51)
  Top 0.203: v40.32,26.43 U$1.13 36.2,26.19 35.4,25.4 31.12,25.4 30.96,25.56 IC12.13 18.73,25.56 18.57,25.4 10.4,25.4 9.68,26.19 9.13,26.75 9.13,29.05 17.15,37.07 17.15,39.93 IC11.14
  Bottom 0.203: v40.32,26.43 39.13,26.43 38.58,26.99 38.58,30.24 39.29,30.96 42.23,30.96 43.1,31.83 50.48,31.83 51.99,33.34 IC3.25
  Bottom 0.406: U1.33 73.34,33.34 72.07,32.07 62.94,32.07 61.67,33.34 IC3.25
D1  (via drill 0.51)
  Top 0.203: 20.24,26.83 17.94,26.83 IC12.14 17.94,27.62 | 20.24,26.83 21.59,26.83 21.83,26.83 23.97,26.83 34.13,26.83 34.77,27.46 U$1.14 40.8,27.46 41.67,28.34 v41.67,29.69 | v18.34,38.58 19.05,39.29 19.05,40.42 IC11.16 | 20.24,26.83 20.24,28.02 20.24,28.73 v20.24,29.92
  Bottom 0.203: v41.67,29.69 50.48,29.69 51.59,30.8 IC3.24 | v18.34,38.58 18.42,38.5 18.42,34.13 18.42,33.26 18.42,32.62 18.42,30.48 18.97,29.92 v20.24,29.92
  Bottom 0.406: IC3.24 61.6,30.8 62.87,29.53 71.91,29.53 73.18,30.8 U1.32
D2  (via drill 0.51)
  Top 0.203: v40.64,28.73 U$1.15 36.67,28.73 36.04,29.37 27.31,29.37 26.99,29.37 23.34,29.37 22.07,30.64 19.45,30.64 | 16.58,27.38 16.51,27.3 | IC12.15 16.58,27.38 | 16.58,27.38 16.67,27.46 16.67,28.89 18.42,30.64 19.45,30.64 | v19.45,30.72 19.45,30.64 | IC11.15 22.45,44.51 18.26,40.32 v18.26,39.93 | v18.26,39.93
  Bottom 0.203: v40.64,28.73 40.8,28.73 42.7,26.83 50.01,26.83 51.44,28.26 59.53,28.26 | IC3.23 58.34,28.26 | 18.26,39.77 v18.26,39.93 18.26,39.77 | 18.26,39.77 19.45,38.58 v19.45,30.72
  Bottom 0.406: U1.31 73.18,28.26 71.91,26.99 71.28,26.99 70.96,26.99 62.55,26.99 61.28,28.26 IC3.23 59.53,28.26
D3  (via drill 0.51)
  Top 0.203: U$1.17 36.2,30 36.83,29.37 40.01,29.37 40.56,29.92 v40.56,30.16 40.56,30.48 40.16,30.88 37.39,30.88 35.8,32.46 15.48,32.46 | 14.13,27.15 IC12.17 14.13,29.37 15.48,30.72 15.48,32.46 | IC11.20 24.19,42.76 20.8,39.37 20.8,38.34 15.48,32.94 15.48,32.46
  Bottom 0.203: IC3.22 51.59,25.72 50.56,24.69 42.15,24.69 41.43,25.4 41.43,27.15 40.96,27.62 39.61,27.62 39.21,28.02 39.21,29.84 39.53,30.16 v40.56,30.16
  Bottom 0.406: IC3.22 61.36,25.72 62.63,24.45 72.39,24.45 73.66,25.72 U1.30
D4  (via drill 0.51)
  Top 0.203: 12.86,27.3 IC12.18 12.86,28.97 12.86,30.24 v14.68,32.07 14.68,31.99 14.68,32.78 20.4,38.5 20.4,39.69 23.83,43.12 IC11.19 | U$1.18 35.4,28.73 | v22.3,29.13 22.7,28.73 U$1.18 | U$1.18 | 35.4,28.73 | 35.4,28.73 v35.8,28.34
  Bottom 0.203: v35.8,28.34 | v35.8,28.34 42.23,21.91 50.48,21.91 51.75,23.18 IC3.21 | v14.68,32.07 16.75,30 17.22,29.53 17.62,29.13 21.11,29.13 21.43,29.13 21.83,29.13 v22.3,29.13
  Bottom 0.406: IC3.21 61.12,23.18 62.39,21.91 72.07,21.91 73.34,23.18 79.85,23.18 80.01,23.02 U1.29
D5  (via drill 0.51)
  Top 0.203: v33.97,27.86 33.58,27.46 25.72,27.46 U$1.19 | IC12.19 11.59,30.24 | 11.59,30.24 v11.59,29.69 11.59,30.24 | v22.3,28.02 22.86,27.46 U$1.19 | U$1.19 | IC11.18 22.75,42.67 19.92,39.85 19.92,38.58 11.59,30.24
  Bottom 0.203: v33.97,27.86 34.05,27.86 34.85,27.86 43.34,19.37 50.64,19.37 51.91,20.64 | v11.59,29.69 13.26,28.02 v22.3,28.02 | IC3.20
  Bottom 0.254: 51.91,20.64 IC3.20
  Bottom 0.406: IC3.20 61.28,20.64 62.55,19.37 72.55,19.37 73.82,20.64 U1.28
D6  (via drill 0.51)
  Top 0.203: v34.85,26.19 U$1.20 23.65,26.19 23.57,26.27 21.19,26.27 21.35,26.27 18.73,26.27 18.26,25.88 10.95,25.88 10.32,26.67 IC12.20 10.32,28.18 10.32,28.97 10.32,29.61 19.45,38.73 19.45,40.08 22.28,42.92 IC11.17
  Bottom 0.203: IC3.19 | IC3.19 52.39,18.1 51.12,16.83 41.91,16.83 34.85,23.89 34.85,24.13 v34.85,26.19
  Bottom 0.406: IC3.19 61.6,18.1 62.87,16.83 72.55,16.83 73.82,18.1 79.85,18.1 79.69,18.1 U1.27
D7  (via drill 0.51)
  Top 0.203: v32.78,33.73 32.46,34.05 25.8,34.05 23.34,36.51 23.34,40.47 IC11.22 | v32.78,33.73
  Bottom 0.203: 59.53,15.56 IC3.18
  Bottom 0.406: IC3.18 61.6,15.56 62.87,14.29 72.55,14.29 73.82,15.56 79.69,15.56 79.85,15.56 U1.26 | 59.53,15.56 52.23,15.56 50.96,14.29 42.86,14.29 41.12,16.03 32.78,24.45 32.78,28.81 32.78,29.77 32.78,31.91 v32.78,33.73
D7RAFL  (via drill 0.51)
  Top 0.203: IC12.21 9.6,25.56 10.32,24.92 U$1.21 35.88,24.92 36.43,25.48 36.51,25.56 40.72,25.56 41.51,26.67 42.31,27.7 42.31,29.21 42.47,29.45 42.47,31.67 41.59,32.54 v40.96,32.54 | IC11.46 35.91,48.06 37.07,46.91 37.07,46.67 37.62,46.12 38.34,46.12 39.53,44.93 v40.8,44.93
  Bottom 0.203: v40.96,32.54 40.96,32.62 40.96,34.29 40.96,35.16 40.96,44.77 v40.8,44.93
FDC_WRITE_IN
  Top 0.203: IC11.53 36.59,53.02 37.47,53.9 38.26,53.9 46.2,45.96 50.96,45.96 51.44,46.43 SV1.3
FDC_WRITE_OUT
  Top 0.203: IC11.54 36.24,53.38 37.23,54.37 38.42,54.37 44.37,48.42 53.42,48.42 53.98,48.97 SV1.6
GND  (via drill 0.51, 0.6, 0.61)  (9 unrouted)
  Top 0.203: 45.56,71.99 D3.A 45.09,71.64 45.09,67.47 46.99,65.56 48.18,65.56 48.91,64.84 50.33,64.84 | 34.08,48.47 35.19,47.36 | 34.08,48.47 35.64,46.91 | 33.34,56.12 33.34,56.2 | 26.91,54.69 27.54,55.32 29.53,57.31 IC11.69 | 28.89,60.8 28.88,60.79 28.53,60.45 | IC11.84 24.29,56.83 24.45,56.83 24.53,56.75 24.92,56.67 25.32,56.2 25.84,55.76 27.38,57.31 27.38,59.37 28.46,60.45 28.53,60.45 | 17.46,52.39 18.89,50.96 20,50.8 | IC11.31 v27.78,45.56 27.54,45.4 26.91,44.77 24.95,42.8 | 75.17,56.52 75.25,63.18 | 28.5,60.48 28.53,60.45 | 33.34,56.12 33.34,56.2 33.41,56.27 | IC11.31 30.8,42.55 | IC11.31 | 24.63,42.49 IC11.21 24.95,42.78 24.95,42.8 | 24.63,42.49 | 24.95,42.8 24.21,42.07 24.21,41.99 | 34.08,48.47 31.07,48.47 v30.88,48.66 | IC6.7 50.32,62.31 | 50.32,62.31 52.04,62.31 IC6.2 | IC6.4 50.33,64.84 | 50.33,64.84 50.32,63.9 50.32,62.63 | 50.32,62.63 50.32,62.31 | IC6.3 50.33,63.57 50.32,62.63 | IC6.1 50.4,61.04 50.32,61.12 50.32,62.31 | 28.81,51.99 28.81,51.83 28.89,52.23 29.45,52.23 33.34,56.12 | 33.34,56.12 | 31.35,50.56 31.19,50.72 | Q1.2 61.29,43.83 62.07,44.61 62.07,49.85 63.18,50.96 64.61,50.96 U1.1 | v47.15,72.55 47.15,73.34 47.47,73.66 Q3.2 | JP1.2
  Top 0.254: v47.15,72.55 46.31,72.55 D3.A
  Top 0.305: U$1.16 36.99,30 35.48,31.51 25.4,31.51 v25.08,31.51
  Top 0.406: C17.- 79.38,56.47 v79.38,54.37 | C4.- 75.17,56.55 v75.17,54.45 | C4.- 70.01,56.55 69.06,57.5 C13.2 | C4.- 74.45,56.55 74.53,56.52 75.17,56.52 | 75.25,63.18 | 75.25,63.18 75.25,56.36 | 75.25,63.18 75.25,66.16 IC2.1 81.24,66.16 81.36,66.28 81.36,68.34 | 79.61,70.64 81.36,70.64 81.36,68.34 | IC1.2 80.25,68.42 80.25,68.34 81.36,68.34 | IC12.16 15.4,29.21 17.7,31.51 v25.08,31.51
  Top 0.61: 25.84,55.76 26.91,54.69 28.81,52.78 28.81,51.83 | v30.88,48.66 31.35,49.05 31.35,50.56 | v25.88,55.72 24.84,56.75 24.53,56.75 | 79.61,70.64 77.07,73.1 | 28.81,51.2 23.81,51.2 20.48,51.2 20,50.8 18.97,50.8 17.94,50.8 16.99,51.28 13.02,51.28 C1.1 12.86,51.28 10.72,51.28 9.92,50.48 | v42.62,45.01 42.62,45.48 37.39,50.72 33.02,50.72 31.19,50.72 30.4,50.72 29.53,50.72 29.29,50.72 28.81,51.2 | 28.81,51.99 28.81,51.2 | 9.92,50.48 9.92,49.93 8.02,49.93 | C6.2 9.92,50.48 | 8.02,49.93 6.27,49.93 JP4.7 | 8.02,49.93
  Top 0.813: C7.2 67.07,50.32 66.36,51.04 64.85,51.04 U1.1
  Bottom 0.203: 41.91,44.29 v42.62,45.01 | 82.63,54.29 81.92,54.29 81.68,54.53 JP2.4 81.6,56.44 | 81.6,56.44 | 29.81,47.59 | 21.35,8.1 C8.2 | 29.81,47.59 | 29.81,47.59 v27.78,45.56 | 29.01,46.79 C5.2 29.73,47.59 29.81,47.59
  Bottom 0.254: IC4.7 56.44,71.68 | IC4.1 48.9,74.83 48.9,71.68 | 53.98,69 53.98,71.68 | 50.24,69.08 50.24,71.68 | IC4.4 52.63,71.68 | 37.53,77.14 37.54,77.15 | 36.26,77.14 36.27,77.15
  Bottom 0.406: v47.15,72.55 47.15,74.61 47.15,76.52 46.51,77.15 37.54,77.15 36.27,77.15 32.23,77.15 31.83,76.76 CON5.22 | 79.3,54.21 79.3,54.29 v79.38,54.37 | 74.53,54.21 74.53,54.29 v75.17,54.45 | 25,31.43 v25.08,31.51 | JP2.4 | JP2.4
  Bottom 0.61: v30.88,48.66 v27.78,45.56 | JP1.2 56.28,2.22 56.28,1.35 | 56.28,1.35 54.37,1.35 54.13,1.43 | 56.28,1.35 75.17,1.35 77.71,1.35 79.14,1.35 80.01,2.22 U1.21 | v25.88,55.72 25.88,54.36 C2.2
  Bottom 0.813: 54.13,1.43 52.23,3.33 25.88,3.33 21.27,7.96 C8.2 | v25.08,31.51 25.08,19.76 18.1,12.78 18.1,9.45 19.45,8.1 21.35,8.1
  Bottom 1.016: 63.34,51.12 U1.1 | 63.34,51.12 62.79,50.56 57.79,45.56 43.18,45.56 41.91,44.29 41.91,38.42 IC3.2 | 63.34,54.29 63.34,51.12 | 63.34,54.29 63.34,71.68 56.44,71.68 53.98,71.68 52.63,71.68 50.24,71.68 48.9,71.68 47.55,71.68 v47.15,72.55 | U1.21 81.6,2.86 82.63,3.89 82.63,54.29 79.3,54.29 74.53,54.29 63.34,54.29
GREENLED  (1 unrouted)
  Top 0.203: 30.74,59.16 35.8,64.21 38.74,64.21 39.37,64.85 R35.1
IIC_CLK  (via drill 0.51)
  Top 0.203: v41.83,74.3 41.83,74.85 43.97,76.99 v64.37,76.99 | IC6.6 45.16,63.58 44.21,62.63 44.21,61.44 41.43,58.66 v38.5,58.66 38.02,58.66 34.5,55.14 IC11.59
  Bottom 0.203: v64.37,76.99 67.07,76.99 67.31,77.15 80.57,77.15 81.28,76.44 81.28,66.6 80.57,65.88 80.09,65.88 78.11,63.9 78.11,59.45 | v41.83,74.3 | v41.83,74.3 40.56,73.03 40.56,65.88 | 40.56,65.88 | 40.56,65.88 40.56,65.41 37.7,62.55 37.7,61.59 38.5,60.72 v38.5,58.66 | 79.22,58.98 | 81.6,58.98
  Bottom 0.254: 81.6,58.98 79.3,58.98 79.22,58.98 R10.1 78.11,59.45
  Bottom 0.406: JP2.3 81.6,58.9 81.6,58.98
IIC_SDA  (via drill 0.51)
  Top 0.203: IC6.5 44.93,64.85 43.74,63.66 43.74,61.83 41.43,59.53 37.39,59.53 v37.07,59.21 37.07,58.42 34.14,55.49 IC11.60
  Top 0.254: v41.51,76.04 43.42,77.87 v64.93,77.87 65.25,77.87
  Bottom 0.203: v41.51,76.04 40.56,76.04 39.45,74.93 39.45,65.01 37.07,62.63 v37.07,59.21 | 81.12,65.41 80.49,65.41 79.06,63.98 R9.1
  Bottom 0.254: 81.12,65.41 81.99,66.28 82.07,76.6 80.8,77.87 66.83,77.87 66.12,77.87 65.17,77.87 v64.93,77.87 | R9.1 81.68,61.52
  Bottom 0.406: 81.68,61.52 | 81.68,61.52 JP2.2
N$2
  Top 0.203: Q1.1 58.19,43.91 R2.2
N$7
  Top 0.203: Q1.3 R4.2 | R4.2
N$8
  Top 0.406: R39.1 49.29,67.31 SG3.+
N$11
  Top 0.203: Q3.3 51.04,73.89 51.04,72.39 50.56,71.91 48.66,71.91 46.99,70.25 46.12,70.25 45.64,69.77 45.64,68.02 47.55,66.12 54.37,66.12 55.96,64.53 D2.A 57.91,63.14 58.26,62.79 58.26,61.99 R3.1
  Top 0.406: SG3.- 58.66,74.61 Q3.3
N$36  (1 unrouted)
  Bottom 0.406: IC3.27 61.75,38.42 63.02,37.15 70.33,37.15 76.68,43.5 79.69,43.5 80.09,43.5
N$41
  Top 0.254: R12.1 72.31,75.8 73.5,76.99 75.72,76.99 75.72,76.91 JP3.4
  Bottom 0.203: 77.15,75.49 JP3.4
  Bottom 0.254: IC4.6 55.17,76.44 55.25,76.44 55.64,76.83 61.36,76.83 65.09,73.1 67.07,73.1 68.26,74.3 75.8,74.3 JP3.4
N$42
  Top 0.254: R11.1 72.47,73.5 JP3.2
  Bottom 0.203: 52.39,77.95 61.44,77.95 63.5,75.8 | JP3.2 | 74.45,75.64 JP3.2 | 63.5,75.8 | 63.5,75.8 64.85,74.45 67.07,74.45 68.18,75.56 JP3.2
  Bottom 0.254: 52.39,77.95 51.36,76.92 IC4.3
N$43  (via drill 0.51)
  Top 0.254: v61.04,68.42 v64.77,68.42
  Bottom 0.254: IC4.9 55.17,70.41 55.48,70.72 59.69,70.72 61.04,69.37 v61.04,68.42 | v64.77,68.42 64.85,68.42 69.45,73.03 JP3.1 74.61,73.03 R14.1
N$44  (via drill 0.51)
  Top 0.254: v55.48,66.36 56.04,66.36 56.91,65.48 v64.93,65.48
  Bottom 0.203: 78.82,69.05 78.5,69.22 73.66,69.22
  Bottom 0.254: IC4.11 52.63,67.23 53.5,66.36 v55.48,66.36 | v64.93,65.48 69.93,65.48 73.66,69.22 | R13.1 78.82,69.05
  Bottom 0.406: JP3.5 79.69,73.03 R13.1
N$86
  Top 0.203: 43.34,68.02 R37.2
  Top 0.254: 43.34,68.02 C3.1
N$96
  Top 0.203: D3.C 45.37,75.76 45.32,75.49 46.36,75.56 | 43.34,74.93 | 43.34,74.93 C3.2
  Top 0.254: 43.34,74.93 43.89,75.49 45.32,75.49 | Q3.1 48.26,75.56 46.36,75.56
N$158
  Top 0.254: R32.2 32.7,70.25 30.56,72.39 30.56,74.53 CON5.20
N$168
  Top 0.254: R33.2 34.93,69.22 34.93,69.29 31.83,72.39 CON5.21
N$174
  Top 0.254: R20.2 5.79,68.82 6.19,69.22 7.94,69.22 8.97,70.25 10.24,70.25 12.3,72.31 13.81,72.31 14.05,72.55 CON5.7
N$175
  Top 0.254: R21.2 8.02,68.42 9.05,69.45 10.24,69.45 12.38,71.6 14.76,71.6 15.32,72.15 15.32,74.53 CON5.8
N$180
  Top 0.254: R22.2 10.24,68.58 12.46,70.8 15.72,70.8 16.59,71.68 CON5.9
N$181
  Top 0.203: R23.2 12.54,68.02
  Top 0.254: 12.54,68.02 12.54,68.9 13.81,70.17 15.88,70.17 17.94,72.23 17.94,74.45 CON5.10
N$182
  Top 0.254: R24.2 14.68,68.98 15.24,69.53 16.43,69.53 19.13,72.23 CON5.11
N$183
  Top 0.254: R25.2 16.91,68.98 20.32,72.39 20.32,74.61 CON5.12
N$184
  Top 0.254: R26.2 19.13,69.93 21.67,72.47 CON5.13
N$185
  Top 0.254: R27.2 21.35,70.41 CON5.15
N$186
  Top 0.254: R36.2 41.59,72.87 37.31,77.15 36.2,77.15 36.12,77.23 35.64,76.76 35.64,74.53 CON5.23
N$187
  Top 0.203: 25.72,71.75 25.72,75.09
  Top 0.254: R28.2 23.81,69.85 25.72,71.75 | 25.72,75.09 25,75.8 CON5.16
N$188
  Top 0.254: R29.2 26.04,71.2 26.75,71.91 CON5.17
N$189
  Top 0.254: R30.2 28.26,71.28 28.02,71.52 28.02,74.53 CON5.18
N$190
  Top 0.254: R31.2 30.48,70.8 29.29,71.99 CON5.19
N$191
  Top 0.254: R35.2 39.37,73.34 CON5.26
N$192
  Top 0.254: R34.2 37.15,73.03 CON5.25
OERAM  (via drill 0.51)  (1 unrouted)
  Top 0.203: IC12.24 14.29,21.75 14.92,21.11 U$1.24 29.21,21.11 30.08,21.11 v30.24,21.11 | 36.94,49.1 38.1,47.94 38.42,47.62 v39.21,46.83
  Bottom 0.203: v30.24,21.11 30.24,21.83 29.92,22.15 28.89,23.18 28.89,35.56 28.97,35.64 30.72,37.39 35.16,41.83 38.1,41.83 38.89,42.62 38.89,44.21 38.89,45.8 39.21,46.12 v39.21,46.83
PHI2  (via drill 0.51)
  Top 0.203: 29.17,41.32 IC11.27 29.22,41.35 38.1,32.54 v39.53,32.54
  Bottom 0.203: 59.77,40.96 IC3.28 50.24,40.96 46.36,37.07 42.94,37.07 42.15,36.27 42.15,32.46 41.43,31.75 40.01,31.75 39.53,32.23 v39.53,32.54
  Bottom 0.254: 59.77,40.96 59.69,41.04
  Bottom 0.406: U1.39 79.77,48.58 79.85,48.58 76.28,48.58 69.93,42.23 60.96,42.23 IC3.28
R/W  (via drill 0.51)
  Top 0.203: v32.7,34.85 26.11,34.85 23.89,37.07 23.89,40.32 IC11.23
  Bottom 0.203: IC3.26 53.82,35.88 50.24,32.31 42.62,32.31 41.67,31.35 37.7,31.35 34.21,34.85 v32.7,34.85
  Bottom 0.406: IC3.26 61.99,35.88 63.26,34.61 63.34,34.61 63.66,34.61 71.76,34.61 73.03,35.88 U1.34
RA8
  Top 0.203: IC12.27 13.81,17.94 14.45,17.3 U$1.27 | U$1.27 | U$1.27 34.69,17.3 35.32,17.94 41.35,17.94 42.55,16.75 46.2,16.75 47.15,17.7 47.15,31.51 46.36,32.31 43.26,32.31 41.75,33.81 38.1,33.81 IC11.29
RA9
  Top 0.203: IC12.26 14.05,19.21 14.68,18.57 U$1.26 | IC11.7 19.58,47.36 14.29,42.07 14.29,38.5 4.37,28.5 4.37,20.95 6.11,19.21 IC12.26 | IC12.26
RA10  (via drill 0.51)
  Top 0.203: IC12.23 14.45,23.02 15.08,22.38 25.24,22.38 25.4,22.23 25.56,22.38 U$1.23 | IC11.41 37.47,42.94 v38.02,42.94 | v28.34,22.38 U$1.23 | U$1.23
  Bottom 0.203: v38.02,42.94 35.64,42.94 35.24,42.55 30.48,37.78 29.53,36.83 28.42,35.72 28.34,35.64 28.34,26.04 v28.34,22.38
RA11
  Top 0.203: IC12.25 14.21,20.48 14.84,19.84 U$1.25 33.1,19.84 | 33.1,19.84 | 33.1,19.84 33.26,19.84 33.89,20.48 41.2,20.48 42.62,21.91 45.96,21.91 46.59,22.54 46.59,31.11 45.88,31.83 43.1,31.83 41.59,33.34 37.86,33.34 IC11.28
RA12  (via drill 0.51)
  Top 0.203: v34.13,15.08 34.45,14.76 U$1.4 40.56,14.76 41.75,13.57 41.75,8.02 42.94,6.83 47.39,6.83 47.55,6.99 49.53,8.97 49.53,13.41 49.53,14.68 49.53,15.8 49.53,31.27 49.53,34.21 48.26,35.48 46.36,37.39 41.91,37.39 38.81,37.39 38.58,37.39 38.89,37.39 38.18,37.39 32.36,43.13 IC11.34 | IC12.4 17.94,13.34 18.1,13.18 v20.56,13.18
  Bottom 0.203: v34.13,15.08 32.23,13.18 31.83,13.18 23.5,13.18 21.75,13.18 21.51,13.18 21.19,13.18 v20.56,13.18 | v34.13,15.08
RA13
  Top 0.203: 25.65,15.94 25.72,15.88 | U$1.28 25.65,15.94 | 25.65,15.94 25.56,16.03 | IC12.28 12.38,16.67 12.78,16.67 | 12.78,16.67 17.46,16.67 18.1,16.03 U$1.28 | U$1.28 | 12.78,16.67 6.19,16.67 3.57,19.29 3.57,28.89 13.49,38.89 13.49,44.77 16.67,47.94 16.75,48.02 IC11.2
RA14
  Top 0.203: 17.94,15.4 19.05,14.37 19.05,14.29 19.29,14.13 28.65,14.13 29.29,13.49 U$1.3 | 17.94,15.4 | 8.41,15.4 IC12.29 | IC12.29 9.37,15.4 10,16.03 17.3,16.03 17.94,15.4 | 8.43,15.41 8.49,15.48 | IC12.29 8.43,15.41 | 8.41,15.4 6.67,15.4 5.24,16.83 3.18,18.89 3.18,29.13 6.11,32.07 7.78,33.73 13.1,39.05 13.1,45.09 16.19,48.18 16.52,48.5 IC11.1 | 8.41,15.4 8.43,15.41
RA15
  Top 0.203: IC12.3 16.67,13.49 | IC11.97 16.67,55.24 4.84,55.24 2.86,53.26 2.78,18.49 6.67,14.61 | IC12.3 16.67,11.99 17.15,11.51 20.56,11.51 22.54,13.49 U$1.30 | U$1.30 | IC12.3 16.67,15.16 16.35,15.48 10.4,15.48 9.13,14.21 7.78,14.21 7.06,14.21 6.67,14.61 | 6.67,14.61
RA16  (via drill 0.51)
  Top 0.203: 15.4,13.65 IC12.2 15.4,11.91 15.4,11.35 15.64,11.11 v15.95,10.79 17.3,10.79 20.8,10.79 22.23,12.22 U$1.31 | v5.95,13.57 4.84,14.68 3.49,16.03 2.38,17.14 2.38,53.34 3.33,54.29 4.68,55.64 16.99,55.64 IC11.96 | U$1.31
  Bottom 0.203: v5.95,13.57 7.62,11.91 14.84,11.91 v15.95,10.79
RA17
  Top 0.203: IC11.95 17.22,56.04 4.45,56.04 1.98,53.58 1.98,30.72 1.98,16.35 7.22,11.11 9.13,11.11 10.32,11.11 | IC12.30 10.32,11.11 | 10.32,11.11 10.32,10.16 12.62,7.86 27.62,7.86 31.99,12.22 U$1.2 | U$1.2
RA18  (via drill 0.51)
  Top 0.203: IC12.1 14.13,10.08 v14.13,10.16 | IC11.94 17.62,56.43 16.91,56.44 4.21,56.44 1.59,53.82 1.59,15.8 10.08,7.3 10.87,7.3 v11.51,7.3 13.65,7.3 28.26,7.3 31.91,10.95 U$1.1 | U$1.1
  Bottom 0.203: v14.13,10.16 14.13,9.37 12.07,7.3 v11.51,7.3
READY_IN
  Top 0.203: IC11.58 34.86,54.78 37.07,56.99 R1.2 40.64,56.91 40.64,54.05 44.85,49.85 SV1.2
READY_IN_OUT
  Top 0.203: IC11.52 | IC11.52 37.7,53.42 38.1,53.42 46.04,45.48 53.1,45.48 53.98,46.28 SV1.5
REDLED  (1 unrouted)
  Top 0.203: R36.1 41.59,64.69 40.56,63.66 35.96,63.66 32.62,60.33 32.62,59.61 31.37,58.35 | 31.37,58.35
RESET  (via drill 0.51)  (1 unrouted)
  Top 0.203: U1.40 79.93,51.2 | 17.9,52.66 17.82,52.66 17.07,53.42 v15.8,53.42 15.63,53.26 C1.2 | JP1.1
  Top 0.254: v44.45,44.29 44.45,44.61 38.26,50.8 v38.26,51.67 | JP1.1 59.13,3.65 59.69,4.21 81.36,4.21 82.47,5.32 82.63,49.45 80.96,51.12 U1.40
  Bottom 0.203: v44.45,44.29 44.37,44.45 | 38.26,53.02 v38.26,51.67
  Bottom 0.254: v38.26,51.67 37.47,51.67 31.09,57.99 30.24,58.82 29.53,59.53 28.5,60.56 25.56,60.56 23.3,58.3 20.72,58.34 v15.8,53.42 | CON5.24 35.64,74.53 35.64,59.45 38.26,56.83 38.26,53.02
  Bottom 0.406: IC3.1 | IC3.1 v44.45,44.29 63.5,44.29 63.82,44.77 69.85,44.77 76.2,51.12 79.97,51.12 | 79.97,51.12 79.97,51.16 | U1.40 79.97,51.12
  Bottom 0.61: v44.45,44.29
RPM_OUT
  Top 0.203: SV1.8 R4.1
SPEED_OUT  (via drill 0.51)
  Top 0.203: R2.1 46.43,43.89 v42.55,47.78 | v15.8,45.48 15.8,46.35 16.59,47.16 16.83,47.39 16.99,47.55 IC11.3
  Bottom 0.203: v42.55,47.78 36.04,47.78 30.64,42.55 25.8,42.55 22.86,45.48 v15.8,45.48
TCK  (via drill 0.51)
  Top 0.203: IC11.48 36.56,48.77 35.8,49.53 v33.5,49.53
  Bottom 0.203: v33.5,49.53 32.54,49.53 30.24,49.53 26.67,49.53 25.56,48.42 21.11,48.42 12.7,48.42 8.65,52.47 7.14,52.47 6.67,52.47 JP4.8
TDI  (via drill 0.51)
  Top 0.203: IC11.45 35.55,47.71 36.59,46.67 36.59,46.51 v37.94,45.16
  Bottom 0.203: v37.94,45.16 37.23,45.16 33.58,41.51 14.61,41.51 12.94,39.85 12.86,39.77 JP4.3
TDO  (via drill 0.51)
  Top 0.203: IC11.83 22.38,59.45 22.07,59.45 v21.75,59.69 | v16.35,50.09 16.35,49.05 12.62,45.32 12.62,39.13 10.72,37.23 JP4.2
  Bottom 0.203: 20.64,59.69 14.84,53.9 14.84,52.63 | 20.64,59.69 | 20.64,59.69 v21.75,59.69
  Bottom 0.254: v16.35,50.09 16.35,51.12 16.19,51.28 | 16.19,51.28 | 16.19,51.28 14.84,52.63
TMS  (via drill 0.51)  (1 unrouted)
  Top 0.203: 36.28,48.42 | 36.28,48.42 37.54,47.15 37.86,47.15 v37.94,47.07
  Bottom 0.203: v37.94,47.07 37.31,46.43 36.35,45.48 35.72,44.85 33.97,43.1 33.26,42.39 32.94,42.07 29.85,42.07 24.13,42.07 22.86,42.07 21.83,42.07 14.76,42.07 11.67,45.09 11.43,45.32 11.19,45.56 10.56,46.2 9.29,47.39 7.54,47.39 6.19,47.39 JP4.6
TURBO_SPEED_IN  (via drill 0.51)
  Top 0.203: v16.91,46.43 16.91,46.77 IC11.4
  Bottom 0.203: SV1.7 56.2,47.31 54.93,48.58 35.96,48.58 30.24,43.02 26.27,43.02 22.86,46.43 v16.91,46.43
VCC  (via drill 0.51, 0.6)  (6 unrouted)
  Top 0.203: v23.26,9.68 23.42,10.87 23.42,10.95 | 78.18,64.14 77.31,64.14 77.31,64.06 76.28,64.06 | 66.2,73.1 66.28,73.1 | U1.38 | U1.38 | 60.52,60.28 60.17,59.93 58.34,59.93 55.88,59.93 49.85,59.93 48.74,61.04 IC6.8 45.32,61.04 42.47,58.18 R1.1 42.55,56.91
  Top 0.254: R12.2 66.28,75.8 | R11.2 66.28,73.5 | 79.61,77.95
  Top 0.305: v47.78,67.94 47.78,68.5 48.58,69.29 R39.2
  Top 0.406: 23.42,10.95 U$1.32 | v23.26,9.68 22.7,9.13 13.41,9.13 12.86,9.68 IC12.32 | v77.95,65.33 77.47,65.25 77.47,63.58 | 78.9,67.47 IC1.1 | 78.9,67.47 78.9,69.37 80.17,69.37 80.2,69.41 | 80.2,69.41 80.25,69.45 | 80.2,69.41 IC1.3 | 78.9,67.47 78.9,69.77 77.95,70.72 76.68,70.72 74.85,70.72 | 66.28,71.6 72.79,71.6 73.5,70.73 IC2.3 | C17.+ 77.47,63.5 77.55,63.58 | R1.1 42.54,56.91 42.55,56.91 | D2.C 55.88,59.74 55.88,59.93 | R3.2 58.34,59.93
  Top 0.61: R39.2 49.61,69.69 50.17,69.69 | 80.08,46.05 U1.38 | 66.68,47.62 66.68,44.37 66.65,44.37 65.78,43.5 U1.4 | v23.26,9.68 23.26,10.72 23.42,10.87 | 79.61,77.95 JP3.6
  Top 0.813: U1.38 72.39,46.04 71.68,46.04 70.17,47.55 | 60.33,61.99 61.12,62.79 65.48,62.79 66.28,63.58 66.28,69.69 | U1.2 65.72,48.58 66.68,47.62 66.75,47.55 70.17,47.55 | v50.48,34.21 v50.48,6.91 | 60.33,61.99 60.33,60.48 60.52,60.28 60.88,59.93 61.67,59.93 62.15,59.45 62.15,56.83 63.1,55.88 64.93,55.88 | 60.33,61.99 | 66.28,69.69 66.28,71.6 66.28,73.5 66.28,75.8 66.28,77.15 67.07,77.95 68.34,77.95 79.61,77.95 81.2,77.95 82.23,76.91 82.23,64.53 JP2.1 81.2,63.5 77.47,63.5 | 70.17,47.55 70.17,50.16 C7.1 70.01,53.58 69.85,53.74 69.85,53.82 67.79,55.88 64.93,55.88 | 50.17,69.69 66.28,69.69 | U1.6 66.04,38.42 66.75,37.7 66.75,34.21 65.88,33.34 U1.8 | 64.93,55.88 D1.C
  Bottom 0.203: 75.88,61.44 75.8,61.12
  Bottom 0.254: R9.2 | 79.45,66.91 R13.2 | R15.2 45.64,64.61 46.36,63.9 48.82,63.9 49.29,64.37 R16.2
  Bottom 0.305: IC4.14 48.82,67.94 48.42,67.31 | 48.42,67.31 v47.78,67.94 | 48.42,67.31 49.29,66.44 R16.2
  Bottom 0.406: R10.2 75.81,61.36 75.88,61.44 | 75.8,61.12 75.8,61.83 75.8,62.79 77.95,64.93 v77.95,65.33 78.34,65.72 79.06,65.72 79.69,66.36 R13.2 | 75.89,61.52 R9.2 | R14.2 77.47,67.39 77.95,66.91 79.45,66.91
  Bottom 0.61: 21.43,9.68 21.75,9.68 | 21.75,9.68 v23.26,9.68 | C8.1 21.51,9.92 21.75,9.68 | 23.26,9.6 v23.26,9.68 | v23.26,9.68
  Bottom 0.813: U1.38 76.84,46.04 69.22,38.42 U1.6 63.5,39.69 55.96,39.69 v50.48,34.21 49.61,33.34 IC3.4 | v50.48,6.91 49.37,5.79 27.07,5.79 23.26,9.6
WERAM  (via drill 0.51)
  Top 0.203: U$1.29 v31.04,14.76 31.67,14.13 40.4,14.13 40.72,13.81 40.72,13.41 40.72,13.18 40.4,12.86 31.59,12.86 27.23,8.49 12.94,8.49 11.59,9.84 IC12.31 | IC12.31 11.59,13.49 | IC11.50 37.36,49.4 38.71,48.05 39.13,47.62 39.53,47.62 39.77,47.39 40.01,47.15 40.4,46.75 v40.4,46.2 | IC12.31
  Bottom 0.203: v31.04,14.76 31.04,18.34 31.04,21.75 29.45,23.34 29.45,35.4 35.32,41.27 38.26,41.27 38.74,41.75 38.81,41.83 39.37,42.39 39.37,45.32 39.93,46.2 v40.4,46.2
YELLOWLED  (1 unrouted)
  Top 0.203: 36.83,66.04 R34.1 37.07,66.04 37.15,65.96 37.15,65.17 37.15,64.77 35.64,64.77 30.31,59.44 30.23,59.44
(copper drawn outside any net)
  shapes: Top area x2

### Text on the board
Top: 65C02 | 1050
Dimension: QUARZ- | LOCH
text: 22.03.2011: Korrekturen: | WE/RAM_ROM_A15 Kurzschluss durch DK beseitigt | VCC_IO an 3.3V anstatt 5V verbunden | Summer war verpolt, nun richtig | 28.03.2011: Bauteilwerte in Silscreen eingetragen, | 100nF an Reset eingebaut | 15.07.2013: LM1117-3,3 als Alternative eingebaut | Schutzdiode eingebaut! Wichtig! | BC847 | Turbo | -> | Centr. | Track-/Density-Display/Config | VREG1 | 100nF | 10R | LM1117 | 3,3V | LP2985-3,3 | 560E or 470E | VREG2 | I2C | 4.7ÂµF | 10ÂµF | 24C02 | 100nF | 100nF | JTAG | 4K53 | 8 x I/O | BC847 | MEGA | MEGA | MEGA | MEGA | MEGA | SPEEDY | SPEEDY | SPEEDY | SPEEDY | 1050 | 1050 | 1050 | 1050 | 39F040 | 512KB SRAM | RESET | (C)2011 mega-hz | (C)2014 ABBUC & MR & GA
